FUNCTION "FC_GRP_82_R12" : VOID
TITLE =GROUP =82_R12
VERSION : 0.1


VAR_TEMP
  CL : "UDT_CABINET";	//CABINET LOCAL
  CR : "UDT_CABINET";	//CABINET REMOTE
  RelError : BOOL ;	//ERROR RELEASE
  RelErrorCL : BOOL ;	//ERROR RELEASE FROM CABINET LOCAL
  RelErrorCR : BOOL ;	//ERROR RELEASE FROM CABINET REMOTE
  RelControl : BOOL ;	//CONTROL RELEASE
  RelControlCL : BOOL ;	//CONTROL RELEASE FROM CABINET LOCAL
  RelControlCR : BOOL ;	//CONTROL RELEASE FROM CABINET REMOTE
  ErrorConfirm : BOOL ;	//ERROR CONFIRM
  AutoOn : BOOL ;	//AUTOMATIC ON
  AutoOff : BOOL ;	//AUTOMATIC OFF
  RelAuto : BOOL ;	//AUTOMATIC RELEASE
  TempSetpoint : REAL ;
  LAMP_ON : BOOL ;
  Speed_Pump_Hz : REAL ;
END_VAR
BEGIN
NETWORK
TITLE =GLOBAL SIGNALS
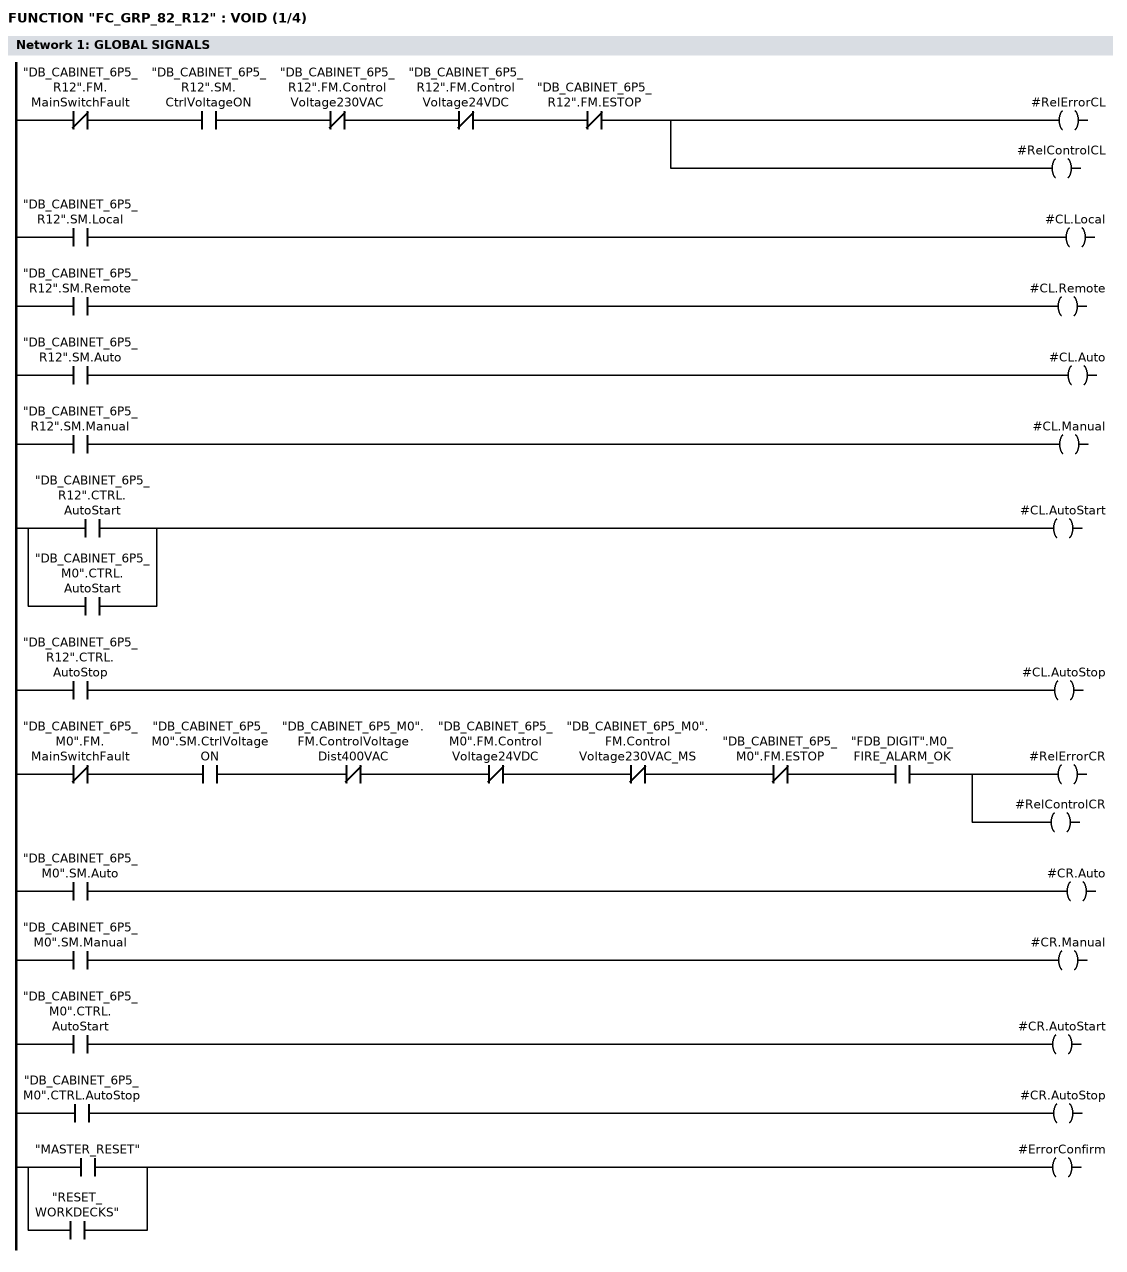
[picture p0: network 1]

      UN    "DB_CABINET_6P5_R12".FM.MainSwitchFault;
      U     "DB_CABINET_6P5_R12".SM.CtrlVoltageON;
      UN    "DB_CABINET_6P5_R12".FM.ControlVoltage230VAC;
      UN    "DB_CABINET_6P5_R12".FM.ControlVoltage24VDC;
      UN    "DB_CABINET_6P5_R12".FM.ESTOP;
      =     #RelErrorCL;
      =     #RelControlCL;

      U     "DB_CABINET_6P5_R12".SM.Local;
      =     #CL.Local;
      U     "DB_CABINET_6P5_R12".SM.Remote;
      =     #CL.Remote;
      U     "DB_CABINET_6P5_R12".SM.Auto;
      =     #CL.Auto;
      U     "DB_CABINET_6P5_R12".SM.Manual;
      =     #CL.Manual;
      U     "DB_CABINET_6P5_R12".CTRL.AutoStart;
      O     "DB_CABINET_6P5_M0".CTRL.AutoStart;
      =     #CL.AutoStart;
      U     "DB_CABINET_6P5_R12".CTRL.AutoStop;
      =     #CL.AutoStop;


      UN    "DB_CABINET_6P5_M0".FM.MainSwitchFault;
      U     "DB_CABINET_6P5_M0".SM.CtrlVoltageON;
      UN    "DB_CABINET_6P5_M0".FM.ControlVoltageDist400VAC;
      UN    "DB_CABINET_6P5_M0".FM.ControlVoltage24VDC;
      UN    "DB_CABINET_6P5_M0".FM.ControlVoltage230VAC_MS;
      UN    "DB_CABINET_6P5_M0".FM.ESTOP;
      U     "FDB_DIGIT".M0_FIRE_ALARM_OK;
      =     #RelErrorCR;
      =     #RelControlCR;

      U     "DB_CABINET_6P5_M0".SM.Auto;
      =     #CR.Auto;
      U     "DB_CABINET_6P5_M0".SM.Manual;
      =     #CR.Manual;
      U     "DB_CABINET_6P5_M0".CTRL.AutoStart;
      =     #CR.AutoStart;
      U     "DB_CABINET_6P5_M0".CTRL.AutoStop;
      =     #CR.AutoStop;


      U     "MASTER_RESET";
      O     "RESET_WORKDECKS";
      =     #ErrorConfirm;

NETWORK
TITLE =GENERAL ERROR AND WARNING
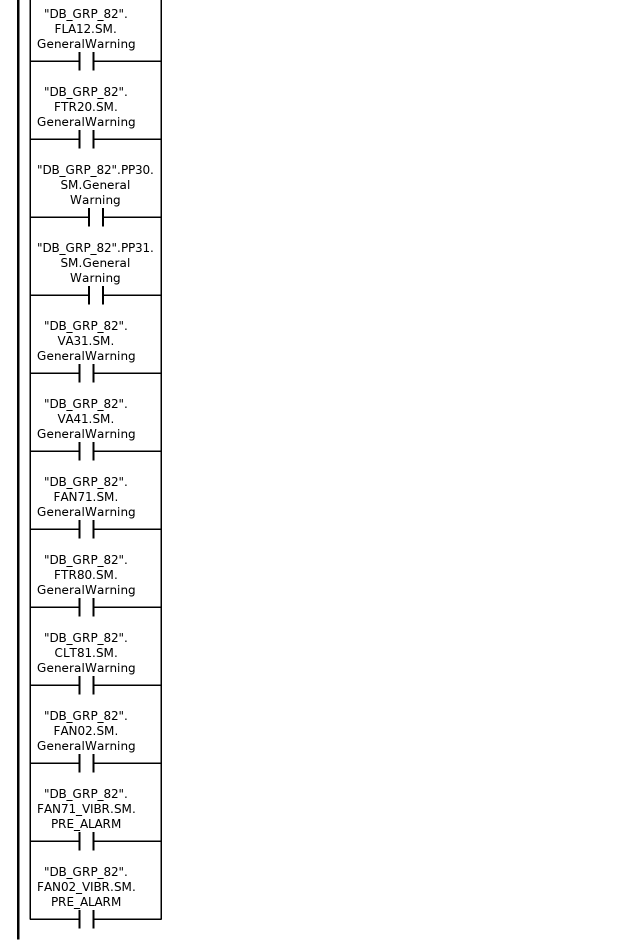
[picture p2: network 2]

      U     "DB_GRP_82".FLA11.SM.GeneralError;
      O     "DB_GRP_82".FLA12.SM.GeneralError;
      O     "DB_GRP_82".FTR20.SM.GeneralError;
      O     "DB_GRP_82".PP30.SM.GeneralError;
      O     "DB_GRP_82".PP31.SM.GeneralError;
      O     "DB_GRP_82".VA31.SM.GeneralError;
      O     "DB_GRP_82".VA41.SM.GeneralError;
      O     "DB_GRP_82".FAN71.SM.GeneralError;
      O     "DB_GRP_82".FTR80.SM.GeneralError;
      O     "DB_GRP_82".CLT81.SM.GeneralError;
      O     "DB_GRP_82".FAN02.SM.GeneralError;
      O     "DB_DIGIT".FM.GRP82_14H2_82FAN02_S32F;
      O     "DB_DIGIT".FM.GRP82_12H2_82FAN71_S32F;
      O     "DB_GRP_82".FAN71_VIBR.SM.GENERAL_ERROR;
      O     "DB_GRP_82".FAN02_VIBR.SM.GENERAL_ERROR;
      O     "DB_DIGIT".FM.GRP82_12H1_82DOO05_S90FA;
      U     "DB_PROG".WorkDecks.SM.WorkDecks2_ASU_ON;
      =     "GENERAL_FAULT_GROUP_82";


      U     "DB_GRP_82".FLA11.SM.GeneralWarning;
      O     "DB_GRP_82".FLA12.SM.GeneralWarning;
      O     "DB_GRP_82".FTR20.SM.GeneralWarning;
      O     "DB_GRP_82".PP30.SM.GeneralWarning;
      O     "DB_GRP_82".PP31.SM.GeneralWarning;
      O     "DB_GRP_82".VA31.SM.GeneralWarning;
      O     "DB_GRP_82".VA41.SM.GeneralWarning;
      O     "DB_GRP_82".FAN71.SM.GeneralWarning;
      O     "DB_GRP_82".FTR80.SM.GeneralWarning;
      O     "DB_GRP_82".CLT81.SM.GeneralWarning;
      O     "DB_GRP_82".FAN02.SM.GeneralWarning;
      O     "DB_GRP_82".FAN71_VIBR.SM.PRE_ALARM;
      O     "DB_GRP_82".FAN02_VIBR.SM.PRE_ALARM;
      =     "WARNING_GROUP_82";


NETWORK
TITLE =GENERAL ERROR 6P5_R12 (FOR LAMP AND HORN)
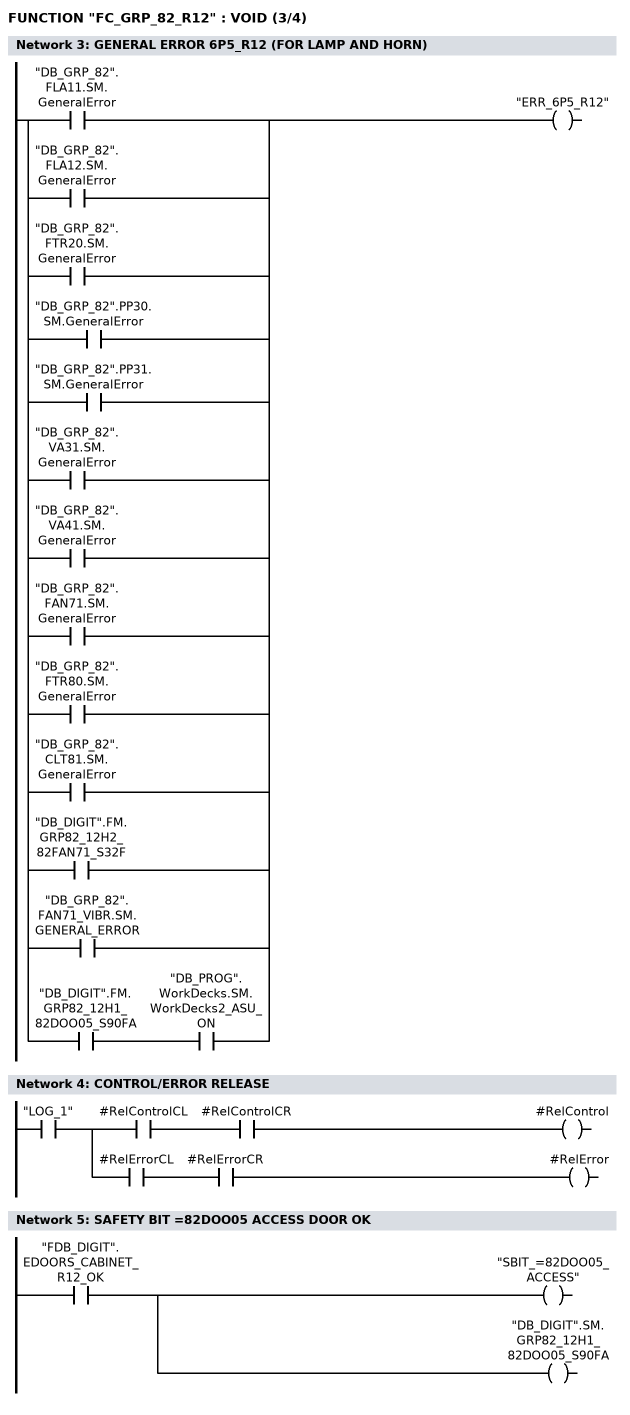
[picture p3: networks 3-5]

      O     "DB_GRP_82".FLA11.SM.GeneralError;
      O     "DB_GRP_82".FLA12.SM.GeneralError;
      O     "DB_GRP_82".FTR20.SM.GeneralError;
      O     "DB_GRP_82".PP30.SM.GeneralError;
      O     "DB_GRP_82".PP31.SM.GeneralError;
      O     "DB_GRP_82".VA31.SM.GeneralError;
      O     "DB_GRP_82".VA41.SM.GeneralError;
      O     "DB_GRP_82".FAN71.SM.GeneralError;
      O     "DB_GRP_82".FTR80.SM.GeneralError;
      O     "DB_GRP_82".CLT81.SM.GeneralError;
      O     "DB_DIGIT".FM.GRP82_12H2_82FAN71_S32F;




      O     "DB_GRP_82".FAN71_VIBR.SM.GENERAL_ERROR;
      O     ;
      U     "DB_DIGIT".FM.GRP82_12H1_82DOO05_S90FA;
      U     "DB_PROG".WorkDecks.SM.WorkDecks2_ASU_ON;
      =     "ERR_6P5_R12";
NETWORK
TITLE =CONTROL/ERROR RELEASE

      U     "LOG_1";
      =     L     16.0;
      U     L     16.0;
      U     #RelControlCL;
      U     #RelControlCR;
      =     #RelControl;
      U     L     16.0;
      U     #RelErrorCL;
      U     #RelErrorCR;
      =     #RelError;
NETWORK
TITLE =SAFETY BIT =82DOO05 ACCESS DOOR OK

      U     "FDB_DIGIT".EDOORS_CABINET_R12_OK;
      =     "SBIT_=82DOO05_ACCESS";
      =     "DB_DIGIT".SM.GRP82_12H1_82DOO05_S90FA;
NETWORK
TITLE ==82DOO05_S90FA ACCESS DOOR OK/FAULT
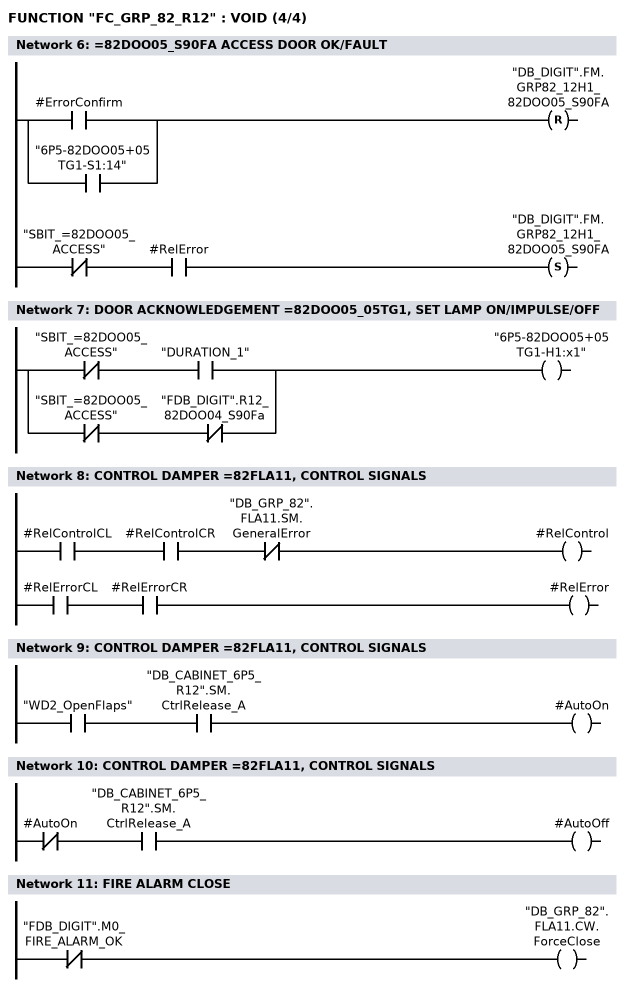
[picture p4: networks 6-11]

      U(    ;
      O     #ErrorConfirm;
      O     "6P5-82DOO05+05TG1-S1:14";
      )     ;
      R     "DB_DIGIT".FM.GRP82_12H1_82DOO05_S90FA;
      UN    "SBIT_=82DOO05_ACCESS";
      U     #RelError;
      S     "DB_DIGIT".FM.GRP82_12H1_82DOO05_S90FA;
      NOP   0;
NETWORK
TITLE =DOOR ACKNOWLEDGEMENT =82DOO05_05TG1, SET LAMP ON/IMPULSE/OFF

      UN    "SBIT_=82DOO05_ACCESS";
      U     "DURATION_1";
      O     ;
      UN    "SBIT_=82DOO05_ACCESS";
      UN    "FDB_DIGIT".R12_82DOO04_S90Fa;
      =     "6P5-82DOO05+05TG1-H1:x1";
NETWORK
TITLE =CONTROL DAMPER =82FLA11, CONTROL SIGNALS

      U     #RelControlCL;
      U     #RelControlCR;
      UN    "DB_GRP_82".FLA11.SM.GeneralError;
      =     #RelControl;

      U     #RelErrorCL;
      U     #RelErrorCR;
      =     #RelError;
NETWORK
TITLE =CONTROL DAMPER =82FLA11, CONTROL SIGNALS

      U     "WD2_OpenFlaps";
      U     "DB_CABINET_6P5_R12".SM.CtrlRelease_A;
      =     #AutoOn;
NETWORK
TITLE =CONTROL DAMPER =82FLA11, CONTROL SIGNALS

      UN    #AutoOn;
      U     "DB_CABINET_6P5_R12".SM.CtrlRelease_A;
      =     #AutoOff;
NETWORK
TITLE =FIRE ALARM CLOSE

      UN    "FDB_DIGIT".M0_FIRE_ALARM_OK;
      =     "DB_GRP_82".FLA11.CW.ForceClose;
NETWORK
TITLE =CONTROL DAMPER =82FLA11

      U     #RelControl;
      =     L     16.0;
      BLD   103;
      U     #RelError;
      =     L     16.1;
      BLD   103;
      U     #AutoOn;
      =     L     16.2;
      BLD   103;
      U     #AutoOff;
      =     L     16.3;
      BLD   103;
      U     "LOG_1";
      =     L     16.4;
      BLD   103;
      U(    ;
      U     "6P5-82FLA11+X-S1c:4";
      L     S5T#1M;
      SE    "T_Delay_Open82FLA11";
      NOP   0;
      NOP   0;
      NOP   0;
      U     "T_Delay_Open82FLA11";
      )     ;
      =     L     16.5;
      BLD   103;
      U(    ;
      U     "6P5-82FLA11+X-S2c:4";
      L     S5T#1M;
      SE    "T_Delay_Close82FLA11";
      NOP   0;
      NOP   0;
      NOP   0;
      U     "T_Delay_Close82FLA11";
      )     ;
      =     L     16.6;
      BLD   103;
      U     #ErrorConfirm;
      =     L     16.7;
      BLD   103;
      CALL "FC_FLAP" (
           REL_CONTROL              := L     16.0,
           REL_ERROR                := L     16.1,
           CL                       := #CL,
           CR                       := #CR,
           AUTO_OPEN                := L     16.2,
           AUTO_CLOSE               := L     16.3,
           FUSE                     := L     16.4,
           LS_OPEN                  := L     16.5,
           LS_CLOSE                 := L     16.6,
           ERROR_CONFIRM            := L     16.7,
           MAX_RUNTIME              := 300,
           OPEN                     := "6P5-82FLA11+X-M1:2",
           CLOSE                    := "6P5-82FLA11+X-M1:3",
           DDB                      := "DB_GRP_82".FLA11);
      NOP   0;
NETWORK
TITLE =CONTROL DAMPER =82FLA12, CONTROL SIGNALS
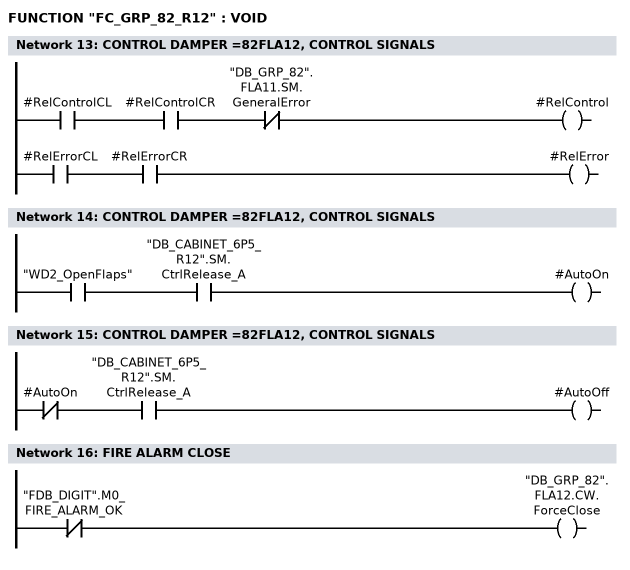
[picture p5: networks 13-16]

      U     #RelControlCL;
      U     #RelControlCR;
      UN    "DB_GRP_82".FLA11.SM.GeneralError;
      =     #RelControl;

      U     #RelErrorCL;
      U     #RelErrorCR;
      =     #RelError;



NETWORK
TITLE =CONTROL DAMPER =82FLA12, CONTROL SIGNALS

      U     "WD2_OpenFlaps";
      U     "DB_CABINET_6P5_R12".SM.CtrlRelease_A;
      =     #AutoOn;
NETWORK
TITLE =CONTROL DAMPER =82FLA12, CONTROL SIGNALS

      UN    #AutoOn;
      U     "DB_CABINET_6P5_R12".SM.CtrlRelease_A;
      =     #AutoOff;
NETWORK
TITLE =FIRE ALARM CLOSE

      UN    "FDB_DIGIT".M0_FIRE_ALARM_OK;
      =     "DB_GRP_82".FLA12.CW.ForceClose;
NETWORK
TITLE =CONTROL DAMPER =82FLA12

      U     #RelControl;
      =     L     16.0;
      BLD   103;
      U     #RelError;
      =     L     16.1;
      BLD   103;
      U     #AutoOn;
      =     L     16.2;
      BLD   103;
      U     #AutoOff;
      =     L     16.3;
      BLD   103;
      U     "LOG_1";
      =     L     16.4;
      BLD   103;
      U(    ;
      U     "6P5-82FLA12+X-S1c:4";
      L     S5T#1M;
      SE    "T_Delay_Open82FLA12";
      NOP   0;
      NOP   0;
      NOP   0;
      U     "T_Delay_Open82FLA12";
      )     ;
      =     L     16.5;
      BLD   103;
      U(    ;
      U     "6P5-82FLA12+X-S2c:4";
      L     S5T#1M;
      SE    "T_Delay_Close82FLA12";
      NOP   0;
      NOP   0;
      NOP   0;
      U     "T_Delay_Close82FLA12";
      )     ;
      =     L     16.6;
      BLD   103;
      U     #ErrorConfirm;
      =     L     16.7;
      BLD   103;
      CALL "FC_FLAP" (
           REL_CONTROL              := L     16.0,
           REL_ERROR                := L     16.1,
           CL                       := #CL,
           CR                       := #CR,
           AUTO_OPEN                := L     16.2,
           AUTO_CLOSE               := L     16.3,
           FUSE                     := L     16.4,
           LS_OPEN                  := L     16.5,
           LS_CLOSE                 := L     16.6,
           ERROR_CONFIRM            := L     16.7,
           MAX_RUNTIME              := 300,
           OPEN                     := "6P5-82FLA12+X-M1:2",
           CLOSE                    := "6P5-82FLA12+X-M1:3",
           DDB                      := "DB_GRP_82".FLA12);
      NOP   0;
NETWORK
TITLE =FILTER MONITOR =82FTR20-B33
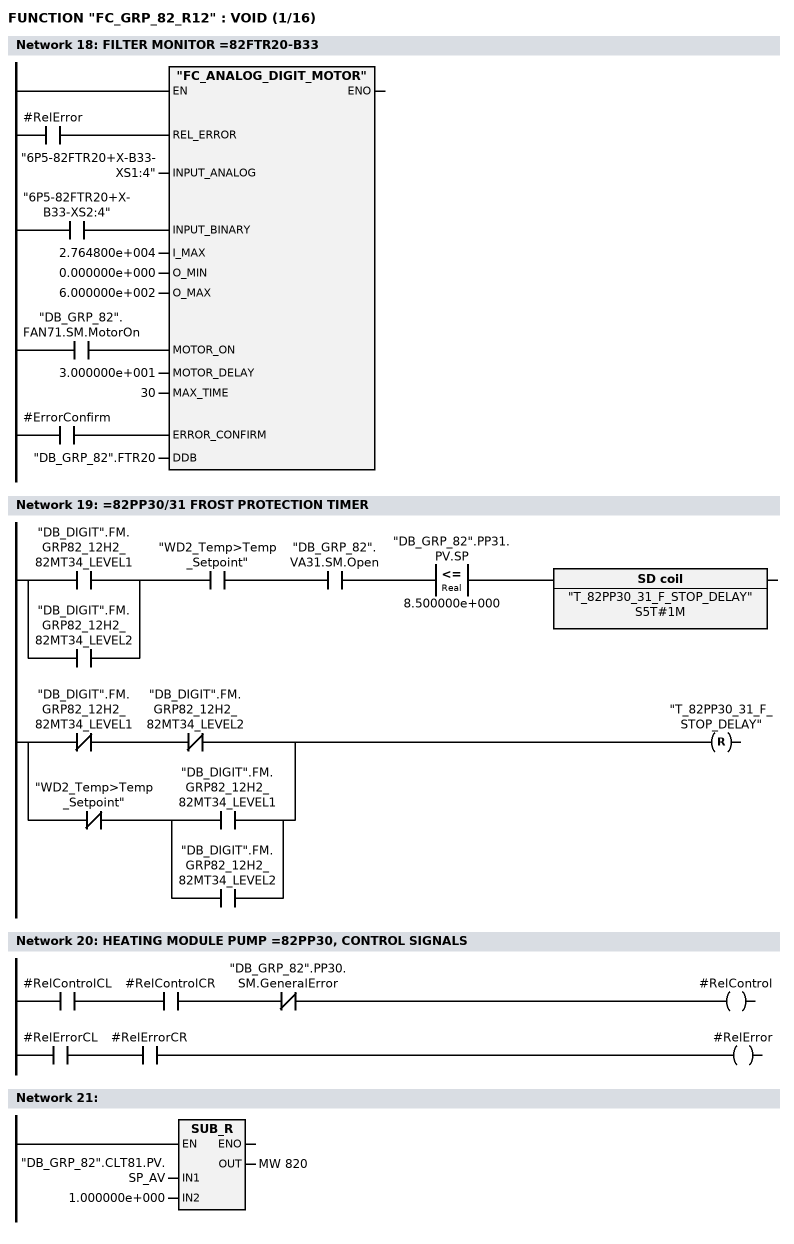
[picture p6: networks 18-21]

      U     #RelError;
      =     L     16.0;
      BLD   103;
      U     "6P5-82FTR20+X-B33-XS2:4";
      =     L     16.1;
      BLD   103;
      U     "DB_GRP_82".FAN71.SM.MotorOn;
      =     L     16.2;
      BLD   103;
      U     #ErrorConfirm;
      =     L     16.3;
      BLD   103;
      CALL "FC_ANALOG_DIGIT_MOTOR" (
           REL_ERROR                := L     16.0,
           INPUT_ANALOG             := "6P5-82FTR20+X-B33-XS1:4",
           INPUT_BINARY             := L     16.1,
           I_MAX                    := 2.764800e+004,
           O_MIN                    := 0.000000e+000,
           O_MAX                    := 6.000000e+002,
           MOTOR_ON                 := L     16.2,
           MOTOR_DELAY              := 3.000000e+001,
           MAX_TIME                 := 30,
           ERROR_CONFIRM            := L     16.3,
           DDB                      := "DB_GRP_82".FTR20);
      NOP   0;
NETWORK
TITLE ==82PP30/31 FROST PROTECTION TIMER

      U(    ;
      O     "DB_DIGIT".FM.GRP82_12H2_82MT34_LEVEL1;
      O     "DB_DIGIT".FM.GRP82_12H2_82MT34_LEVEL2;
      )     ;
      U     "WD2_Temp>Temp_Setpoint";
      U     "DB_GRP_82".VA31.SM.Open;
      U(    ;
      L     "DB_GRP_82".PP31.PV.SP;
      L     8.500000e+000;
      <=R   ;
      )     ;
      L     S5T#1M;
      SE    "T_82PP30_31_F_STOP_DELAY";
      U(    ;
      UN    "DB_DIGIT".FM.GRP82_12H2_82MT34_LEVEL1;
      UN    "DB_DIGIT".FM.GRP82_12H2_82MT34_LEVEL2;
      O     ;
      UN    "WD2_Temp>Temp_Setpoint";
      U(    ;
      O     "DB_DIGIT".FM.GRP82_12H2_82MT34_LEVEL1;
      O     "DB_DIGIT".FM.GRP82_12H2_82MT34_LEVEL2;
      )     ;
      )     ;
      R     "T_82PP30_31_F_STOP_DELAY";
      NOP   0;
      NOP   0;
      NOP   0;
NETWORK
TITLE =HEATING MODULE PUMP =82PP30, CONTROL SIGNALS

      U     #RelControlCL;
      U     #RelControlCR;
      UN    "DB_GRP_82".PP30.SM.GeneralError;
      =     #RelControl;

      U     #RelErrorCL;
      U     #RelErrorCR;
      =     #RelError;

NETWORK
TITLE =

      L     "DB_GRP_82".CLT81.PV.SP_AV;
      L     1.000000e+000;
      -R    ;
      T     MW   820;
      NOP   0;
NETWORK
TITLE =AUTO ON
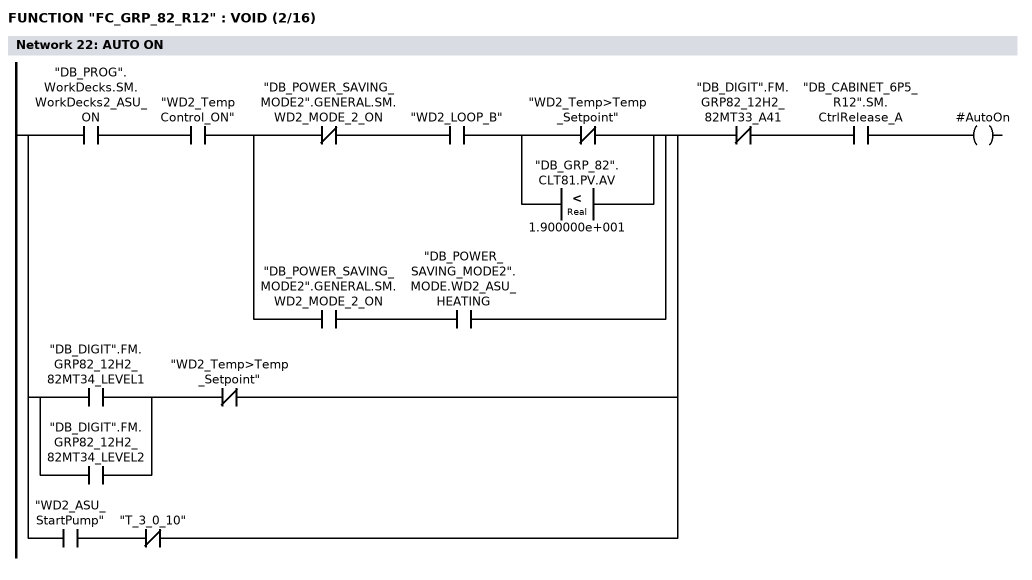
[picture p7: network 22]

      U(    ;
      U     "DB_PROG".WorkDecks.SM.WorkDecks2_ASU_ON;
      U     "WD2_TempControl_ON";
      U(    ;
      UN    "DB_POWER_SAVING_MODE2".GENERAL.SM.WD2_MODE_2_ON;
      U     "WD2_LOOP_B";
      U(    ;
      ON    "WD2_Temp>Temp_Setpoint";
      O(    ;
      L     "DB_GRP_82".CLT81.PV.AV;
      L     1.900000e+001;
      <R    ;
      )     ;
      )     ;
      O     ;
      U     "DB_POWER_SAVING_MODE2".GENERAL.SM.WD2_MODE_2_ON;
      U     "DB_POWER_SAVING_MODE2".MODE.WD2_ASU_HEATING;
      )     ;
      O     ;
      U(    ;
      O     "DB_DIGIT".FM.GRP82_12H2_82MT34_LEVEL1;
      O     "DB_DIGIT".FM.GRP82_12H2_82MT34_LEVEL2;
      )     ;
      UN    "WD2_Temp>Temp_Setpoint";
      O     ;
      U     "WD2_ASU_StartPump";
      UN    "T_3_0_10";
      )     ;
      UN    "DB_DIGIT".FM.GRP82_12H2_82MT33_A41;
      U     "DB_CABINET_6P5_R12".SM.CtrlRelease_A;
      =     #AutoOn;
NETWORK
TITLE =AUTO OFF
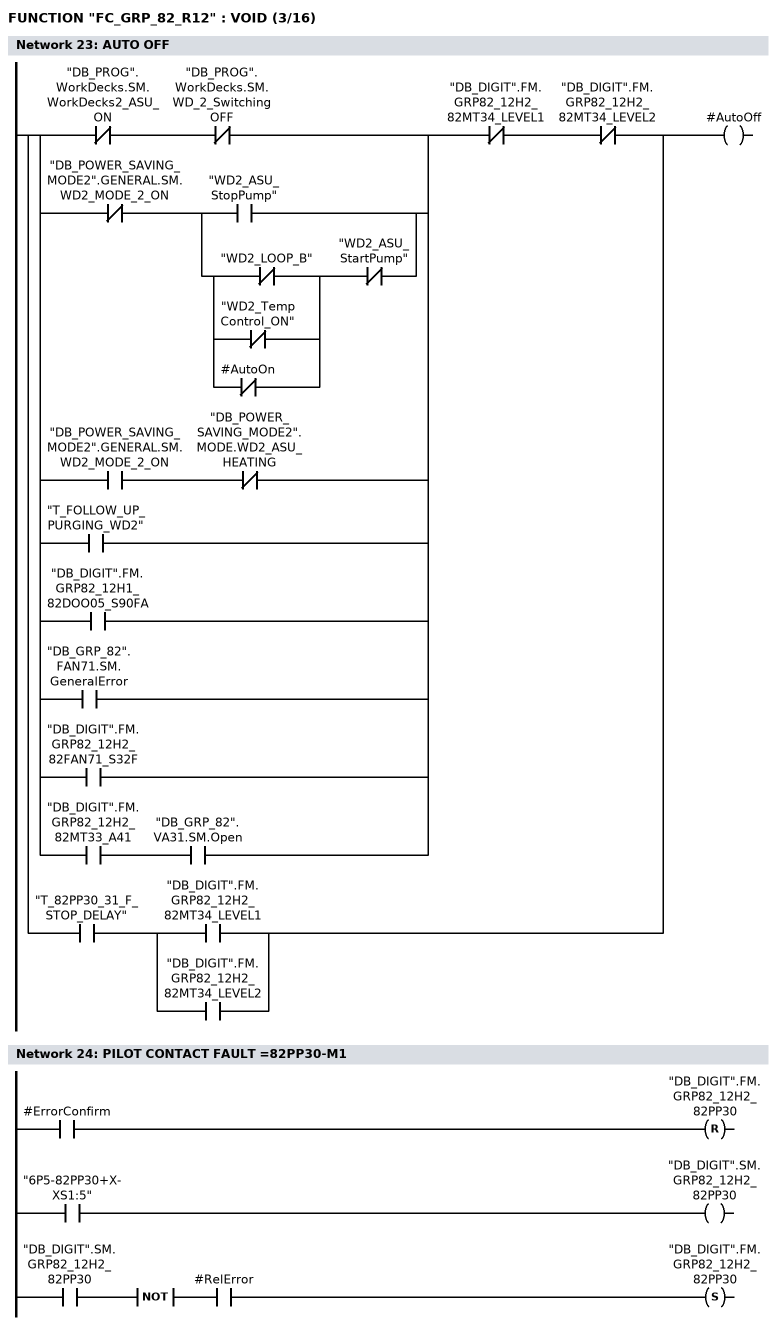
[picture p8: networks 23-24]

      U(    ;
      UN    "DB_PROG".WorkDecks.SM.WorkDecks2_ASU_ON;
      UN    "DB_PROG".WorkDecks.SM.WD_2_SwitchingOFF;
      O     ;
      UN    "DB_POWER_SAVING_MODE2".GENERAL.SM.WD2_MODE_2_ON;
      U(    ;
      O     "WD2_ASU_StopPump";
      O     ;
      U(    ;
      ON    "WD2_LOOP_B";
      ON    "WD2_TempControl_ON";
      ON    #AutoOn;
      )     ;
      UN    "WD2_ASU_StartPump";
      )     ;
      O     ;
      U     "DB_POWER_SAVING_MODE2".GENERAL.SM.WD2_MODE_2_ON;
      UN    "DB_POWER_SAVING_MODE2".MODE.WD2_ASU_HEATING;
      O     "T_FOLLOW_UP_PURGING_WD2";
      O     "DB_DIGIT".FM.GRP82_12H1_82DOO05_S90FA;
      O     "DB_GRP_82".FAN71.SM.GeneralError;
      O     "DB_DIGIT".FM.GRP82_12H2_82FAN71_S32F;
      O     ;
      U     "DB_DIGIT".FM.GRP82_12H2_82MT33_A41;
      U     "DB_GRP_82".VA31.SM.Open;
      )     ;
      UN    "DB_DIGIT".FM.GRP82_12H2_82MT34_LEVEL1;
      UN    "DB_DIGIT".FM.GRP82_12H2_82MT34_LEVEL2;
      O     ;
      U     "T_82PP30_31_F_STOP_DELAY";
      U(    ;
      O     "DB_DIGIT".FM.GRP82_12H2_82MT34_LEVEL1;
      O     "DB_DIGIT".FM.GRP82_12H2_82MT34_LEVEL2;
      )     ;
      =     #AutoOff;
NETWORK
TITLE =PILOT CONTACT FAULT =82PP30-M1

      U     #ErrorConfirm;
      R     "DB_DIGIT".FM.GRP82_12H2_82PP30;
      U     "6P5-82PP30+X-XS1:5";
      =     "DB_DIGIT".SM.GRP82_12H2_82PP30;
      U     "DB_DIGIT".SM.GRP82_12H2_82PP30;
      NOT   ;
      U     #RelError;
      S     "DB_DIGIT".FM.GRP82_12H2_82PP30;
      NOP   0;
NETWORK
TITLE =HEATING MODULE PUMP, =82PP30-M1
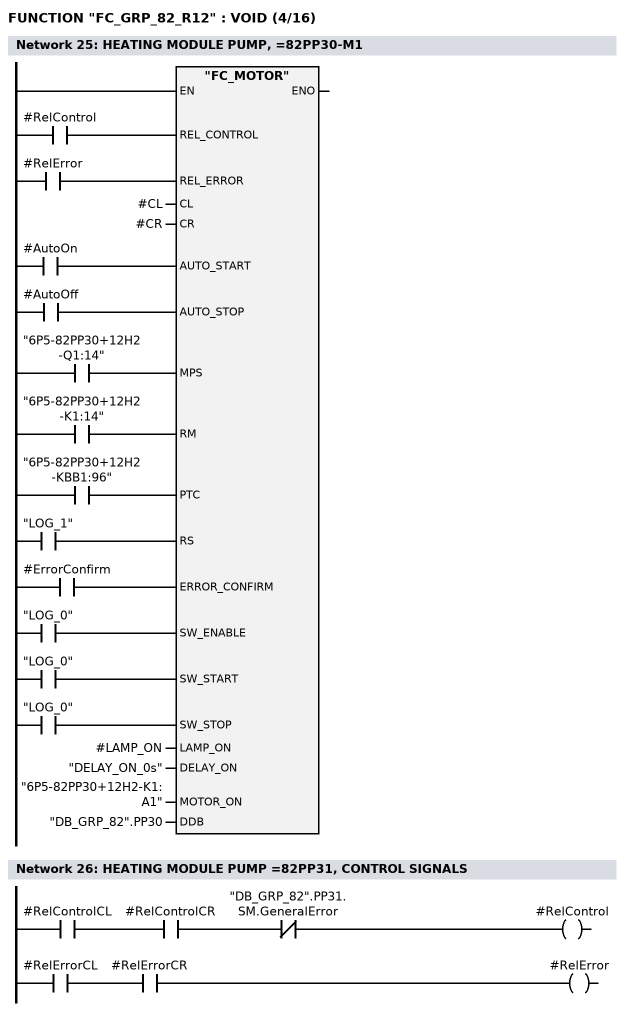
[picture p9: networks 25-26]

      U     #RelControl;
      =     L     16.0;
      BLD   103;
      U     #RelError;
      =     L     16.1;
      BLD   103;
      U     #AutoOn;
      =     L     16.2;
      BLD   103;
      U     #AutoOff;
      =     L     16.3;
      BLD   103;
      U     "6P5-82PP30+12H2-Q1:14";
      =     L     16.4;
      BLD   103;
      U     "6P5-82PP30+12H2-K1:14";
      =     L     16.5;
      BLD   103;
      U     "6P5-82PP30+12H2-KBB1:96";
      =     L     16.6;
      BLD   103;
      U     "LOG_1";
      =     L     16.7;
      BLD   103;
      U     #ErrorConfirm;
      =     L     17.0;
      BLD   103;
      U     "LOG_0";
      =     L     17.1;
      BLD   103;
      U     "LOG_0";
      =     L     17.2;
      BLD   103;
      U     "LOG_0";
      =     L     17.3;
      BLD   103;
      CALL "FC_MOTOR" (
           REL_CONTROL              := L     16.0,
           REL_ERROR                := L     16.1,
           CL                       := #CL,
           CR                       := #CR,
           AUTO_START               := L     16.2,
           AUTO_STOP                := L     16.3,
           MPS                      := L     16.4,
           RM                       := L     16.5,
           PTC                      := L     16.6,
           RS                       := L     16.7,
           ERROR_CONFIRM            := L     17.0,
           SW_ENABLE                := L     17.1,
           SW_START                 := L     17.2,
           SW_STOP                  := L     17.3,
           LAMP_ON                  := #LAMP_ON,
           DELAY_ON                 := "DELAY_ON_0s",
           MOTOR_ON                 := "6P5-82PP30+12H2-K1:A1",
           DDB                      := "DB_GRP_82".PP30);
      NOP   0;
NETWORK
TITLE =HEATING MODULE PUMP =82PP31, CONTROL SIGNALS

      U     #RelControlCL;
      U     #RelControlCR;
      UN    "DB_GRP_82".PP31.SM.GeneralError;
      =     #RelControl;

      U     #RelErrorCL;
      U     #RelErrorCR;
      =     #RelError;



NETWORK
TITLE =AUTO ON
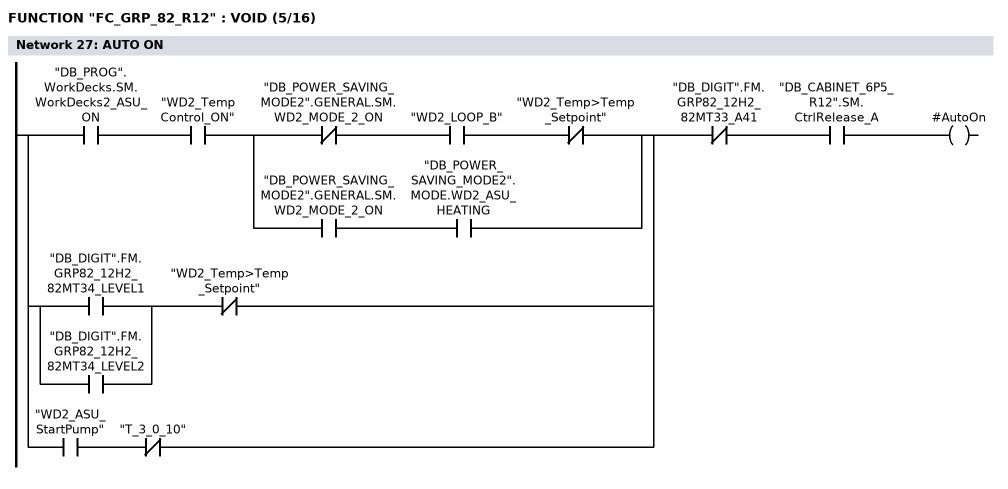
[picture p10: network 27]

      U(    ;
      U     "DB_PROG".WorkDecks.SM.WorkDecks2_ASU_ON;
      U     "WD2_TempControl_ON";
      U(    ;
      UN    "DB_POWER_SAVING_MODE2".GENERAL.SM.WD2_MODE_2_ON;
      U     "WD2_LOOP_B";
      UN    "WD2_Temp>Temp_Setpoint";
      O     ;
      U     "DB_POWER_SAVING_MODE2".GENERAL.SM.WD2_MODE_2_ON;
      U     "DB_POWER_SAVING_MODE2".MODE.WD2_ASU_HEATING;
      )     ;
      O     ;
      U(    ;
      O     "DB_DIGIT".FM.GRP82_12H2_82MT34_LEVEL1;
      O     "DB_DIGIT".FM.GRP82_12H2_82MT34_LEVEL2;
      )     ;
      UN    "WD2_Temp>Temp_Setpoint";
      O     ;
      U     "WD2_ASU_StartPump";
      UN    "T_3_0_10";
      )     ;
      UN    "DB_DIGIT".FM.GRP82_12H2_82MT33_A41;
      U     "DB_CABINET_6P5_R12".SM.CtrlRelease_A;
      =     #AutoOn;
NETWORK
TITLE =AUTO OFF
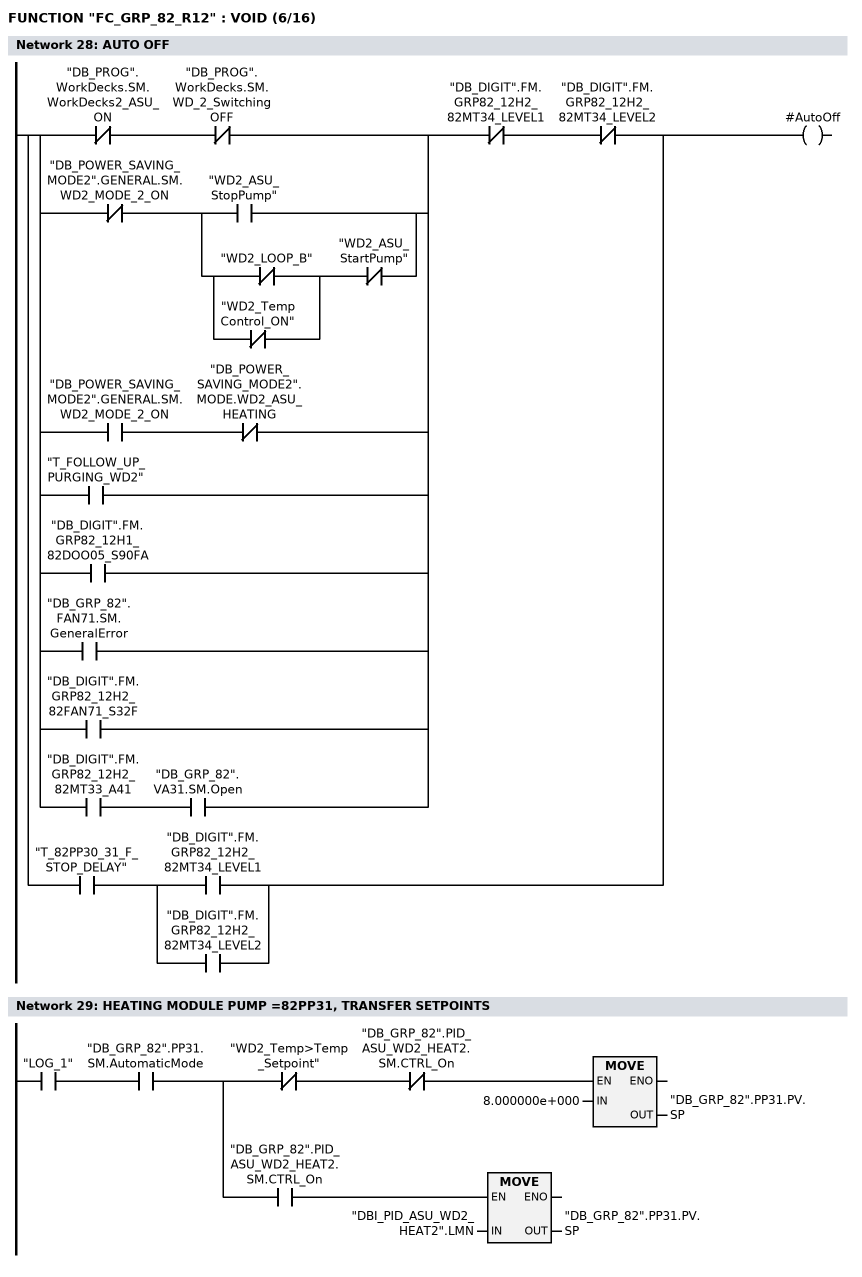
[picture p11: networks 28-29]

      U(    ;
      UN    "DB_PROG".WorkDecks.SM.WorkDecks2_ASU_ON;
      UN    "DB_PROG".WorkDecks.SM.WD_2_SwitchingOFF;
      O     ;
      UN    "DB_POWER_SAVING_MODE2".GENERAL.SM.WD2_MODE_2_ON;
      U(    ;
      O     "WD2_ASU_StopPump";
      O     ;
      U(    ;
      ON    "WD2_LOOP_B";
      ON    "WD2_TempControl_ON";
      )     ;
      UN    "WD2_ASU_StartPump";
      )     ;
      O     ;
      U     "DB_POWER_SAVING_MODE2".GENERAL.SM.WD2_MODE_2_ON;
      UN    "DB_POWER_SAVING_MODE2".MODE.WD2_ASU_HEATING;
      O     "T_FOLLOW_UP_PURGING_WD2";
      O     "DB_DIGIT".FM.GRP82_12H1_82DOO05_S90FA;
      O     "DB_GRP_82".FAN71.SM.GeneralError;
      O     "DB_DIGIT".FM.GRP82_12H2_82FAN71_S32F;
      O     ;
      U     "DB_DIGIT".FM.GRP82_12H2_82MT33_A41;
      U     "DB_GRP_82".VA31.SM.Open;
      )     ;
      UN    "DB_DIGIT".FM.GRP82_12H2_82MT34_LEVEL1;
      UN    "DB_DIGIT".FM.GRP82_12H2_82MT34_LEVEL2;
      O     ;
      U     "T_82PP30_31_F_STOP_DELAY";
      U(    ;
      O     "DB_DIGIT".FM.GRP82_12H2_82MT34_LEVEL1;
      O     "DB_DIGIT".FM.GRP82_12H2_82MT34_LEVEL2;
      )     ;
      =     #AutoOff;
NETWORK
TITLE =HEATING MODULE PUMP =82PP31, TRANSFER SETPOINTS

      U     "LOG_1";
      U     "DB_GRP_82".PP31.SM.AutomaticMode;
      =     L     16.0;
      U     L     16.0;
      UN    "WD2_Temp>Temp_Setpoint";
      UN    "DB_GRP_82".PID_ASU_WD2_HEAT2.SM.CTRL_On;
      SPBNB _001;
      L     8.000000e+000;
      T     "DB_GRP_82".PP31.PV.SP;
_001: NOP   0;
      U     L     16.0;
      U     "DB_GRP_82".PID_ASU_WD2_HEAT2.SM.CTRL_On;
      SPBNB _002;
      L     "DBI_PID_ASU_WD2_HEAT2".LMN;
      T     "DB_GRP_82".PP31.PV.SP;
_002: NOP   0;
NETWORK
TITLE =HEATING MODULE PUMP, =82PP31_M1
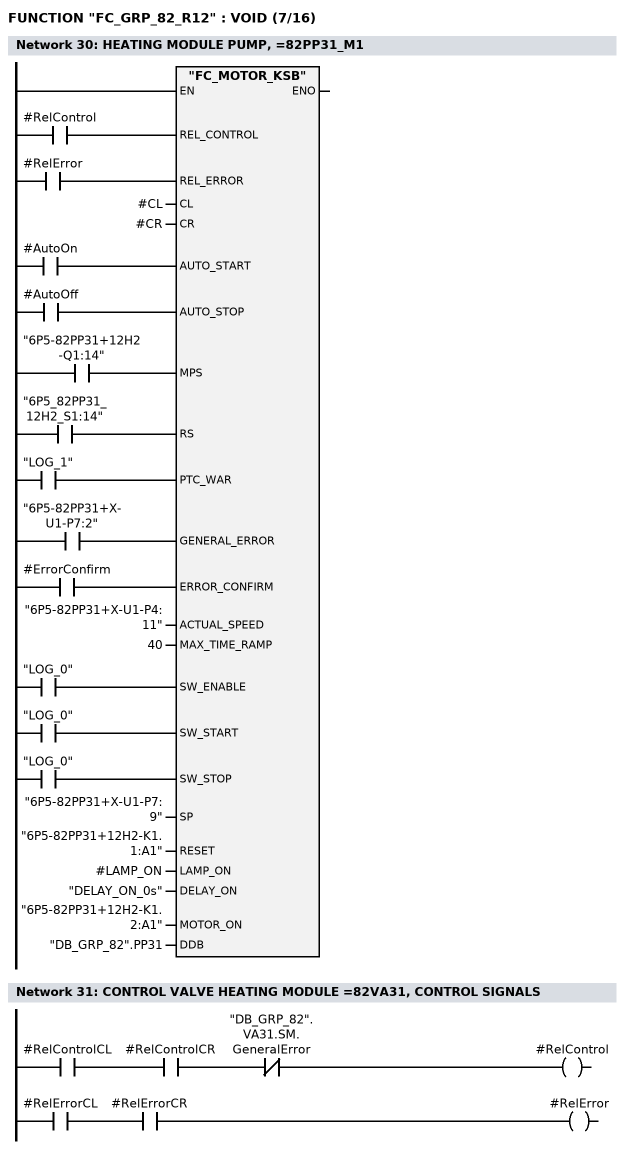
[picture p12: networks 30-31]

      U     #RelControl;
      =     L     16.0;
      BLD   103;
      U     #RelError;
      =     L     16.1;
      BLD   103;
      U     #AutoOn;
      =     L     16.2;
      BLD   103;
      U     #AutoOff;
      =     L     16.3;
      BLD   103;
      U     "6P5-82PP31+12H2-Q1:14";
      =     L     16.4;
      BLD   103;
      U     "6P5_82PP31_12H2_S1:14";
      =     L     16.5;
      BLD   103;
      U     "LOG_1";
      =     L     16.6;
      BLD   103;
      U     "6P5-82PP31+X-U1-P7:2";
      =     L     16.7;
      BLD   103;
      U     #ErrorConfirm;
      =     L     17.0;
      BLD   103;
      U     "LOG_0";
      =     L     17.1;
      BLD   103;
      U     "LOG_0";
      =     L     17.2;
      BLD   103;
      U     "LOG_0";
      =     L     17.3;
      BLD   103;
      CALL "FC_MOTOR_KSB" (
           REL_CONTROL              := L     16.0,
           REL_ERROR                := L     16.1,
           CL                       := #CL,
           CR                       := #CR,
           AUTO_START               := L     16.2,
           AUTO_STOP                := L     16.3,
           MPS                      := L     16.4,
           RS                       := L     16.5,
           PTC_WAR                  := L     16.6,
           GENERAL_ERROR            := L     16.7,
           ERROR_CONFIRM            := L     17.0,
           ACTUAL_SPEED             := "6P5-82PP31+X-U1-P4:11",
           MAX_TIME_RAMP            := 40,
           SW_ENABLE                := L     17.1,
           SW_START                 := L     17.2,
           SW_STOP                  := L     17.3,
           SP                       := "6P5-82PP31+X-U1-P7:9",
           RESET                    := "6P5-82PP31+12H2-K1.1:A1",
           LAMP_ON                  := #LAMP_ON,
           DELAY_ON                 := "DELAY_ON_0s",
           MOTOR_ON                 := "6P5-82PP31+12H2-K1.2:A1",
           DDB                      := "DB_GRP_82".PP31);
      NOP   0;
NETWORK
TITLE =CONTROL VALVE HEATING MODULE =82VA31, CONTROL SIGNALS

      U     #RelControlCL;
      U     #RelControlCR;
      UN    "DB_GRP_82".VA31.SM.GeneralError;
      =     #RelControl;

      U     #RelErrorCL;
      U     #RelErrorCR;
      =     #RelError;
NETWORK
TITLE =AUTO ON
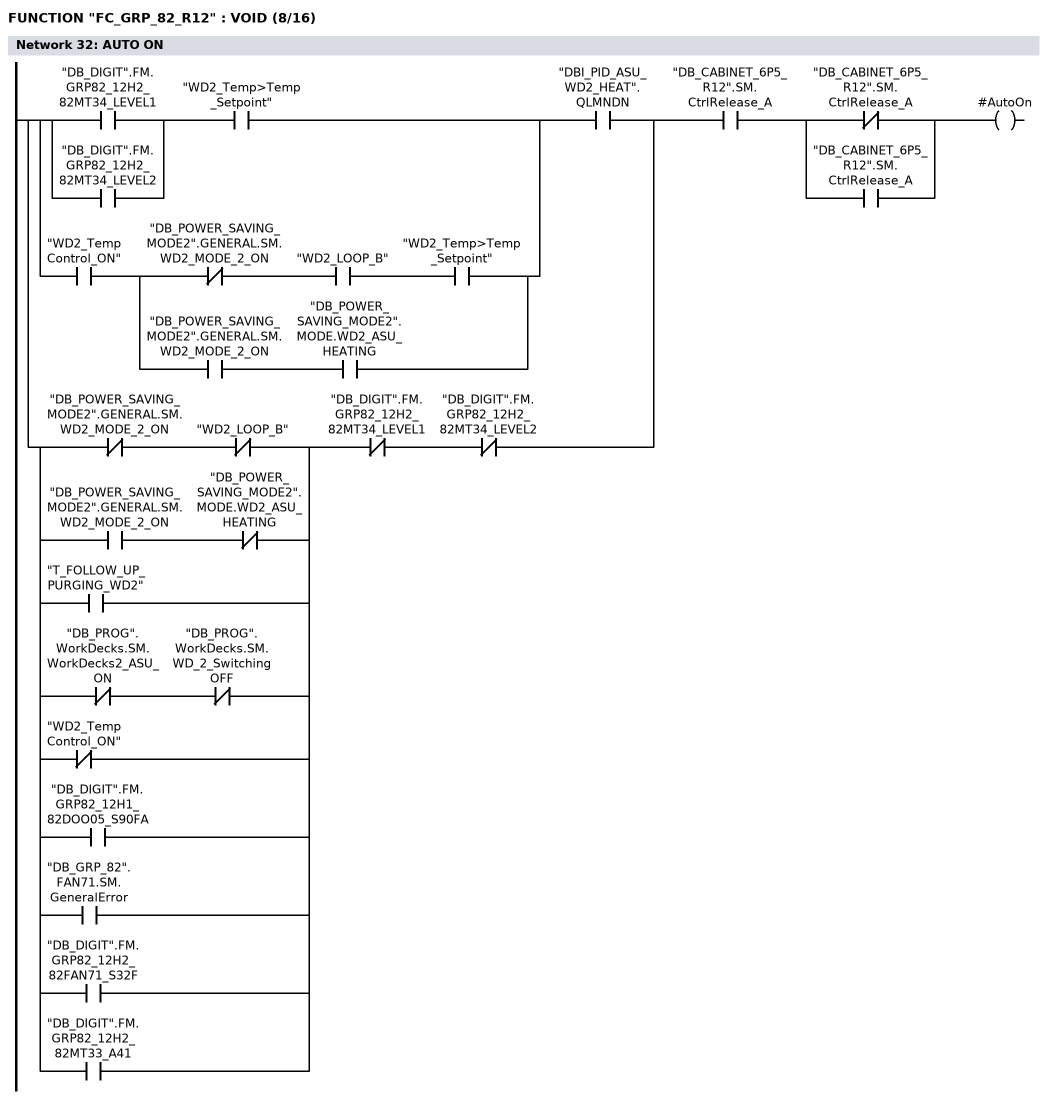
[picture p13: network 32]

      U(    ;
      U(    ;
      U(    ;
      O     "DB_DIGIT".FM.GRP82_12H2_82MT34_LEVEL1;
      O     "DB_DIGIT".FM.GRP82_12H2_82MT34_LEVEL2;
      )     ;
      U     "WD2_Temp>Temp_Setpoint";
      O     ;
      U     "WD2_TempControl_ON";
      U(    ;
      UN    "DB_POWER_SAVING_MODE2".GENERAL.SM.WD2_MODE_2_ON;
      U     "WD2_LOOP_B";
      U     "WD2_Temp>Temp_Setpoint";
      O     ;
      U     "DB_POWER_SAVING_MODE2".GENERAL.SM.WD2_MODE_2_ON;
      U     "DB_POWER_SAVING_MODE2".MODE.WD2_ASU_HEATING;
      )     ;
      )     ;
      U     "DBI_PID_ASU_WD2_HEAT".QLMNDN;
      O     ;
      U(    ;
      UN    "DB_POWER_SAVING_MODE2".GENERAL.SM.WD2_MODE_2_ON;
      UN    "WD2_LOOP_B";
      O     ;
      U     "DB_POWER_SAVING_MODE2".GENERAL.SM.WD2_MODE_2_ON;
      UN    "DB_POWER_SAVING_MODE2".MODE.WD2_ASU_HEATING;
      O     "T_FOLLOW_UP_PURGING_WD2";
      O     ;
      UN    "DB_PROG".WorkDecks.SM.WorkDecks2_ASU_ON;
      UN    "DB_PROG".WorkDecks.SM.WD_2_SwitchingOFF;
      ON    "WD2_TempControl_ON";
      O     "DB_DIGIT".FM.GRP82_12H1_82DOO05_S90FA;
      O     "DB_GRP_82".FAN71.SM.GeneralError;
      O     "DB_DIGIT".FM.GRP82_12H2_82FAN71_S32F;
      O     "DB_DIGIT".FM.GRP82_12H2_82MT33_A41;
      )     ;
      UN    "DB_DIGIT".FM.GRP82_12H2_82MT34_LEVEL1;
      UN    "DB_DIGIT".FM.GRP82_12H2_82MT34_LEVEL2;
      )     ;
      U     "DB_CABINET_6P5_R12".SM.CtrlRelease_A;
      U(    ;
      ON    "DB_CABINET_6P5_R12".SM.CtrlRelease_A;
      O     "DB_CABINET_6P5_R12".SM.CtrlRelease_A;
      )     ;
      =     #AutoOn;
NETWORK
TITLE =AUTO OFF
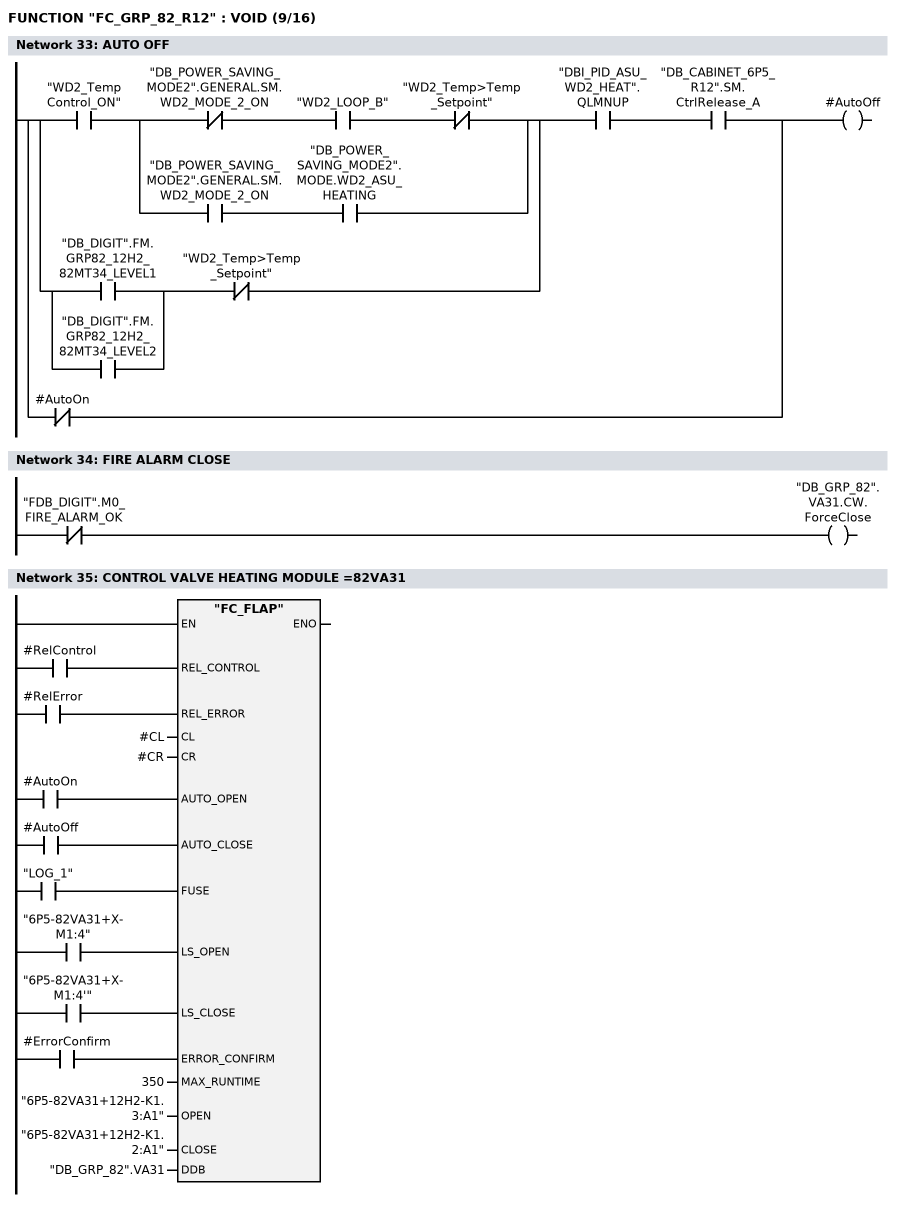
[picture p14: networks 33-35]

      U(    ;
      U     "WD2_TempControl_ON";
      U(    ;
      UN    "DB_POWER_SAVING_MODE2".GENERAL.SM.WD2_MODE_2_ON;
      U     "WD2_LOOP_B";
      UN    "WD2_Temp>Temp_Setpoint";
      O     ;
      U     "DB_POWER_SAVING_MODE2".GENERAL.SM.WD2_MODE_2_ON;
      U     "DB_POWER_SAVING_MODE2".MODE.WD2_ASU_HEATING;
      )     ;
      O     ;
      U(    ;
      O     "DB_DIGIT".FM.GRP82_12H2_82MT34_LEVEL1;
      O     "DB_DIGIT".FM.GRP82_12H2_82MT34_LEVEL2;
      )     ;
      UN    "WD2_Temp>Temp_Setpoint";
      )     ;
      U     "DBI_PID_ASU_WD2_HEAT".QLMNUP;
      U     "DB_CABINET_6P5_R12".SM.CtrlRelease_A;
      ON    #AutoOn;
      =     #AutoOff;
NETWORK
TITLE =FIRE ALARM CLOSE

      UN    "FDB_DIGIT".M0_FIRE_ALARM_OK;
      =     "DB_GRP_82".VA31.CW.ForceClose;
NETWORK
TITLE =CONTROL VALVE HEATING MODULE =82VA31

      U     #RelControl;
      =     L     16.0;
      BLD   103;
      U     #RelError;
      =     L     16.1;
      BLD   103;
      U     #AutoOn;
      =     L     16.2;
      BLD   103;
      U     #AutoOff;
      =     L     16.3;
      BLD   103;
      U     "LOG_1";
      =     L     16.4;
      BLD   103;
      U     "6P5-82VA31+X-M1:4";
      =     L     16.5;
      BLD   103;
      U     "6P5-82VA31+X-M1:4'";
      =     L     16.6;
      BLD   103;
      U     #ErrorConfirm;
      =     L     16.7;
      BLD   103;
      CALL "FC_FLAP" (
           REL_CONTROL              := L     16.0,
           REL_ERROR                := L     16.1,
           CL                       := #CL,
           CR                       := #CR,
           AUTO_OPEN                := L     16.2,
           AUTO_CLOSE               := L     16.3,
           FUSE                     := L     16.4,
           LS_OPEN                  := L     16.5,
           LS_CLOSE                 := L     16.6,
           ERROR_CONFIRM            := L     16.7,
           MAX_RUNTIME              := 350,
           OPEN                     := "6P5-82VA31+12H2-K1.3:A1",
           CLOSE                    := "6P5-82VA31+12H2-K1.2:A1",
           DDB                      := "DB_GRP_82".VA31);
      NOP   0;
NETWORK
TITLE =READ POSITION =82VA31
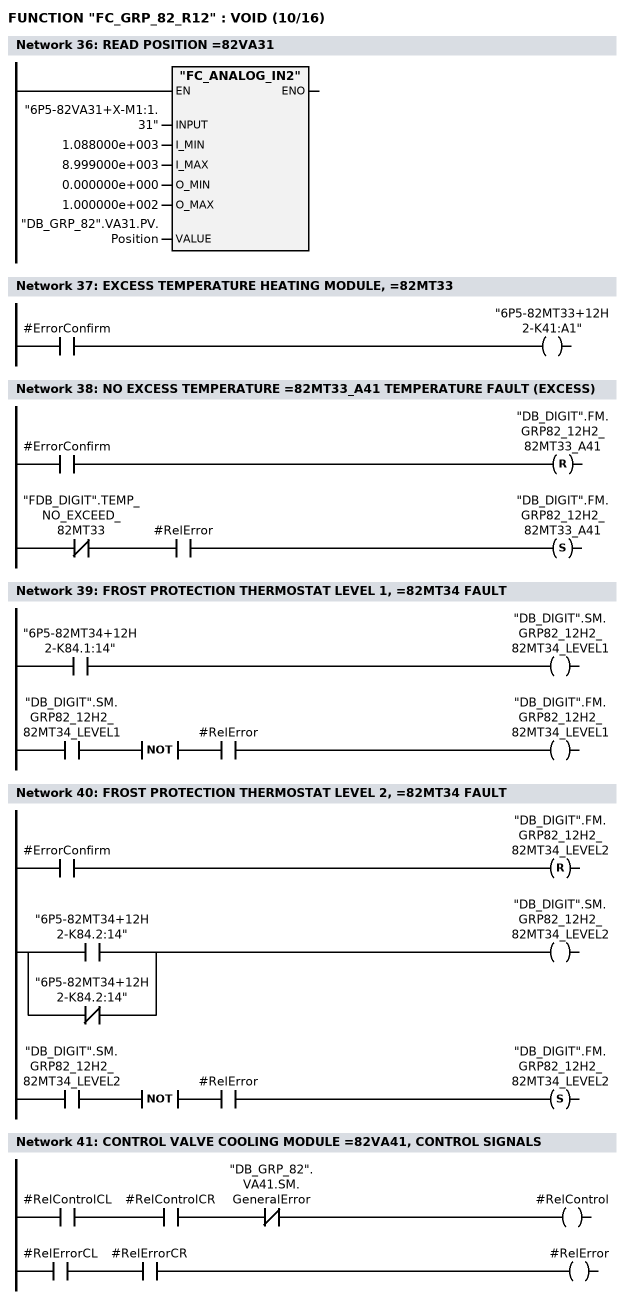
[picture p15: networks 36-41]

      CALL "FC_ANALOG_IN2" (
           INPUT                    := "6P5-82VA31+X-M1:1.31",
           I_MIN                    := 1.088000e+003,
           I_MAX                    := 8.999000e+003,
           O_MIN                    := 0.000000e+000,
           O_MAX                    := 1.000000e+002,
           VALUE                    := "DB_GRP_82".VA31.PV.Position);
      NOP   0;
NETWORK
TITLE =EXCESS TEMPERATURE HEATING MODULE, =82MT33

      U     #ErrorConfirm;
      =     "6P5-82MT33+12H2-K41:A1";
NETWORK
TITLE =NO EXCESS TEMPERATURE =82MT33_A41 TEMPERATURE FAULT (EXCESS)

      U     #ErrorConfirm;
      R     "DB_DIGIT".FM.GRP82_12H2_82MT33_A41;
      UN    "FDB_DIGIT".TEMP_NO_EXCEED_82MT33;
      U     #RelError;
      S     "DB_DIGIT".FM.GRP82_12H2_82MT33_A41;
      NOP   0;
NETWORK
TITLE =FROST PROTECTION THERMOSTAT LEVEL 1, =82MT34 FAULT

      U     "6P5-82MT34+12H2-K84.1:14";
      =     "DB_DIGIT".SM.GRP82_12H2_82MT34_LEVEL1;
      U     "DB_DIGIT".SM.GRP82_12H2_82MT34_LEVEL1;
      NOT   ;
      U     #RelError;
      =     "DB_DIGIT".FM.GRP82_12H2_82MT34_LEVEL1;
NETWORK
TITLE =FROST PROTECTION THERMOSTAT LEVEL 2, =82MT34 FAULT

      U     #ErrorConfirm;
      R     "DB_DIGIT".FM.GRP82_12H2_82MT34_LEVEL2;
      U(    ;
      O     "6P5-82MT34+12H2-K84.2:14";
      ON    "6P5-82MT34+12H2-K84.2:14";
      )     ;
      =     "DB_DIGIT".SM.GRP82_12H2_82MT34_LEVEL2;
      U     "DB_DIGIT".SM.GRP82_12H2_82MT34_LEVEL2;
      NOT   ;
      U     #RelError;
      S     "DB_DIGIT".FM.GRP82_12H2_82MT34_LEVEL2;
      NOP   0;
NETWORK
TITLE =CONTROL VALVE COOLING MODULE =82VA41, CONTROL SIGNALS

      U     #RelControlCL;
      U     #RelControlCR;
      UN    "DB_GRP_82".VA41.SM.GeneralError;
      =     #RelControl;

      U     #RelErrorCL;
      U     #RelErrorCR;
      =     #RelError;


NETWORK
TITLE =RELEASE =82VA41
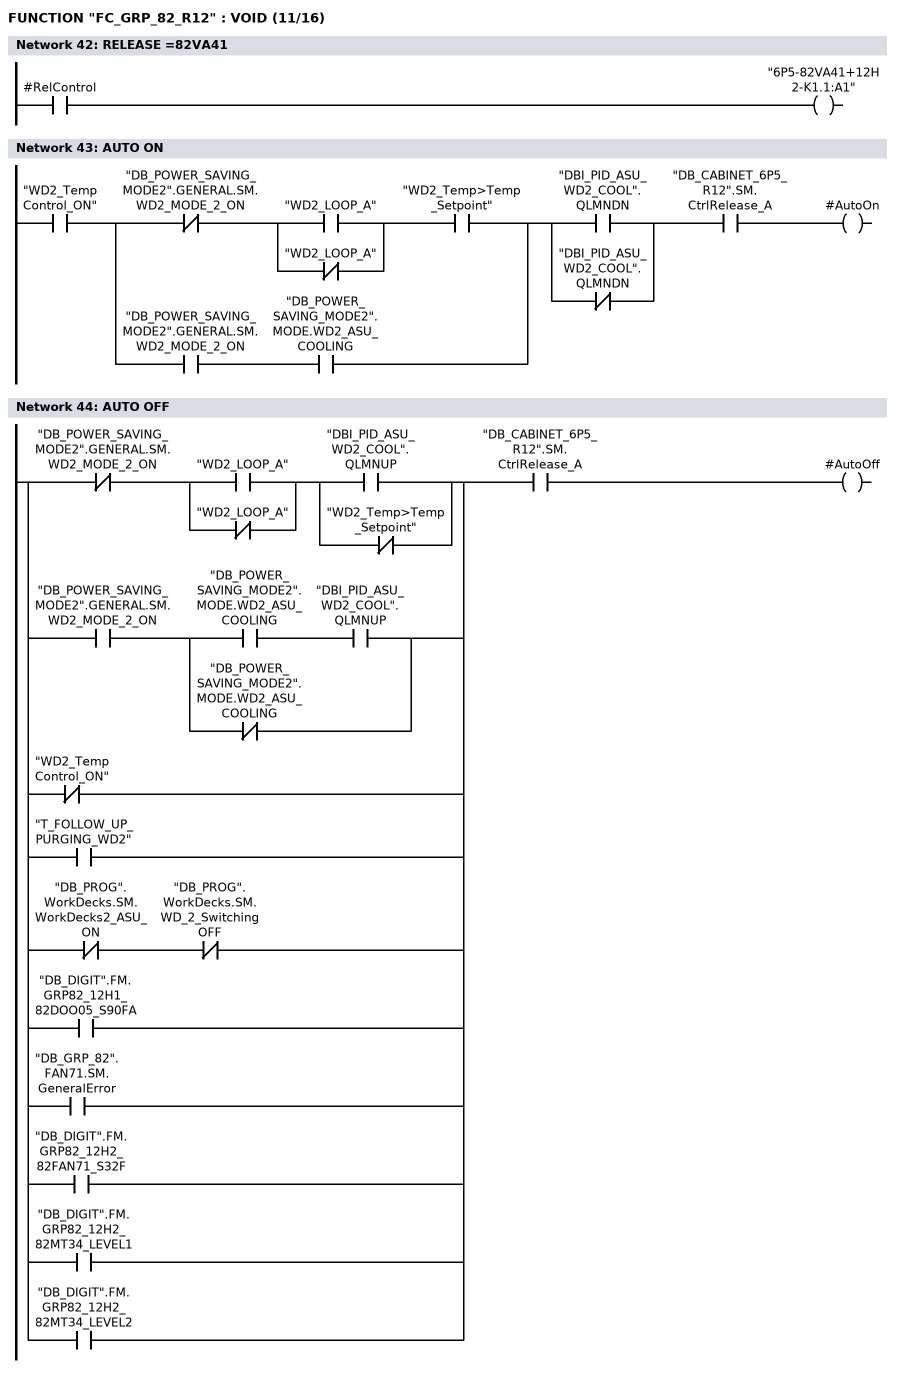
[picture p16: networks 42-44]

      U     #RelControl;
      =     "6P5-82VA41+12H2-K1.1:A1";
NETWORK
TITLE =AUTO ON

      U     "WD2_TempControl_ON";
      U(    ;
      UN    "DB_POWER_SAVING_MODE2".GENERAL.SM.WD2_MODE_2_ON;
      U(    ;
      O     "WD2_LOOP_A";
      ON    "WD2_LOOP_A";
      )     ;
      U     "WD2_Temp>Temp_Setpoint";
      O     ;
      U     "DB_POWER_SAVING_MODE2".GENERAL.SM.WD2_MODE_2_ON;
      U     "DB_POWER_SAVING_MODE2".MODE.WD2_ASU_COOLING;
      )     ;
      U(    ;
      O     "DBI_PID_ASU_WD2_COOL".QLMNDN;
      ON    "DBI_PID_ASU_WD2_COOL".QLMNDN;
      )     ;
      U     "DB_CABINET_6P5_R12".SM.CtrlRelease_A;
      =     #AutoOn;
NETWORK
TITLE =AUTO OFF

      U(    ;
      UN    "DB_POWER_SAVING_MODE2".GENERAL.SM.WD2_MODE_2_ON;
      U(    ;
      O     "WD2_LOOP_A";
      ON    "WD2_LOOP_A";
      )     ;
      U(    ;
      O     "DBI_PID_ASU_WD2_COOL".QLMNUP;
      ON    "WD2_Temp>Temp_Setpoint";
      )     ;
      O     ;
      U     "DB_POWER_SAVING_MODE2".GENERAL.SM.WD2_MODE_2_ON;
      U(    ;
      U     "DB_POWER_SAVING_MODE2".MODE.WD2_ASU_COOLING;
      U     "DBI_PID_ASU_WD2_COOL".QLMNUP;
      ON    "DB_POWER_SAVING_MODE2".MODE.WD2_ASU_COOLING;
      )     ;
      ON    "WD2_TempControl_ON";
      O     "T_FOLLOW_UP_PURGING_WD2";
      O     ;
      UN    "DB_PROG".WorkDecks.SM.WorkDecks2_ASU_ON;
      UN    "DB_PROG".WorkDecks.SM.WD_2_SwitchingOFF;
      O     "DB_DIGIT".FM.GRP82_12H1_82DOO05_S90FA;
      O     "DB_GRP_82".FAN71.SM.GeneralError;
      O     "DB_DIGIT".FM.GRP82_12H2_82FAN71_S32F;
      O     "DB_DIGIT".FM.GRP82_12H2_82MT34_LEVEL1;
      O     "DB_DIGIT".FM.GRP82_12H2_82MT34_LEVEL2;
      )     ;
      U     "DB_CABINET_6P5_R12".SM.CtrlRelease_A;
      =     #AutoOff;
NETWORK
TITLE =FIRE ALARM CLOSE
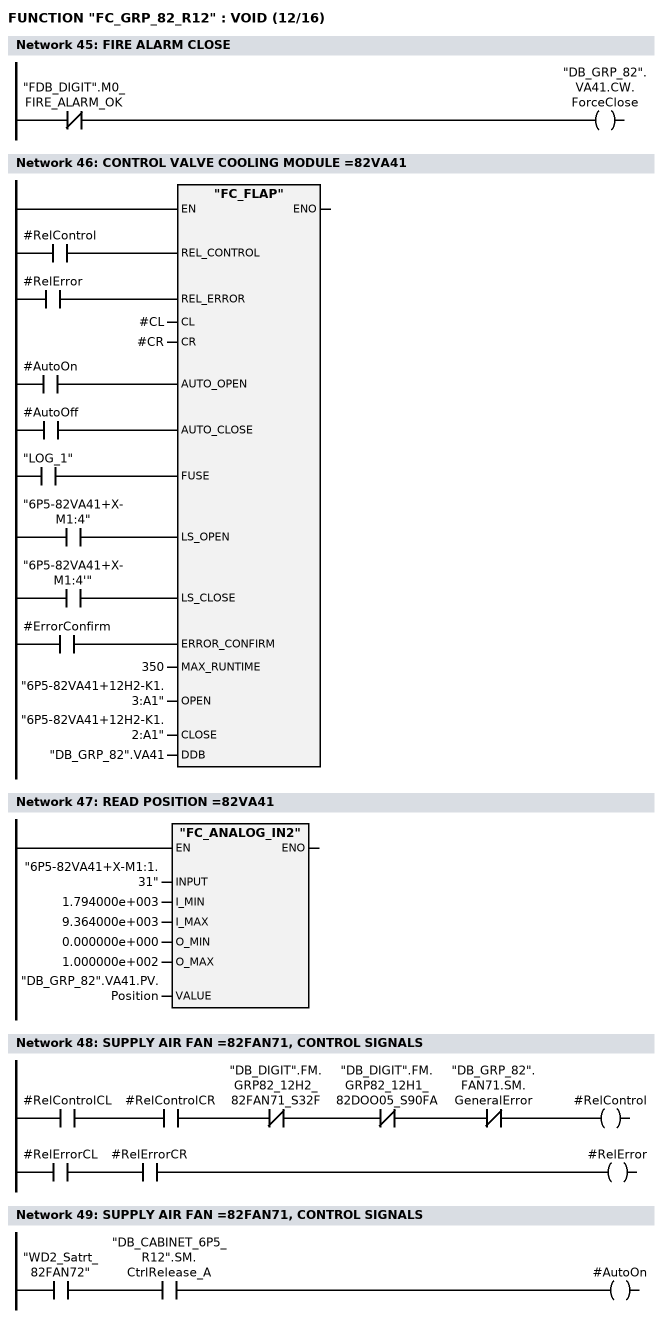
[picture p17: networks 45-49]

      UN    "FDB_DIGIT".M0_FIRE_ALARM_OK;
      =     "DB_GRP_82".VA41.CW.ForceClose;
NETWORK
TITLE =CONTROL VALVE COOLING MODULE =82VA41

      U     #RelControl;
      =     L     16.0;
      BLD   103;
      U     #RelError;
      =     L     16.1;
      BLD   103;
      U     #AutoOn;
      =     L     16.2;
      BLD   103;
      U     #AutoOff;
      =     L     16.3;
      BLD   103;
      U     "LOG_1";
      =     L     16.4;
      BLD   103;
      U     "6P5-82VA41+X-M1:4";
      =     L     16.5;
      BLD   103;
      U     "6P5-82VA41+X-M1:4'";
      =     L     16.6;
      BLD   103;
      U     #ErrorConfirm;
      =     L     16.7;
      BLD   103;
      CALL "FC_FLAP" (
           REL_CONTROL              := L     16.0,
           REL_ERROR                := L     16.1,
           CL                       := #CL,
           CR                       := #CR,
           AUTO_OPEN                := L     16.2,
           AUTO_CLOSE               := L     16.3,
           FUSE                     := L     16.4,
           LS_OPEN                  := L     16.5,
           LS_CLOSE                 := L     16.6,
           ERROR_CONFIRM            := L     16.7,
           MAX_RUNTIME              := 350,
           OPEN                     := "6P5-82VA41+12H2-K1.3:A1",
           CLOSE                    := "6P5-82VA41+12H2-K1.2:A1",
           DDB                      := "DB_GRP_82".VA41);
      NOP   0;
NETWORK
TITLE =READ POSITION =82VA41

      CALL "FC_ANALOG_IN2" (
           INPUT                    := "6P5-82VA41+X-M1:1.31",
           I_MIN                    := 1.794000e+003,
           I_MAX                    := 9.364000e+003,
           O_MIN                    := 0.000000e+000,
           O_MAX                    := 1.000000e+002,
           VALUE                    := "DB_GRP_82".VA41.PV.Position);
      NOP   0;
NETWORK
TITLE =SUPPLY AIR FAN =82FAN71, CONTROL SIGNALS

      U     #RelControlCL;
      U     #RelControlCR;
      UN    "DB_DIGIT".FM.GRP82_12H2_82FAN71_S32F;
      UN    "DB_DIGIT".FM.GRP82_12H1_82DOO05_S90FA;
      UN    "DB_GRP_82".FAN71.SM.GeneralError;
      =     #RelControl;

      U     #RelErrorCL;
      U     #RelErrorCR;
      =     #RelError;



NETWORK
TITLE =SUPPLY AIR FAN =82FAN71, CONTROL SIGNALS

      U     "WD2_Satrt_82FAN72";
      U     "DB_CABINET_6P5_R12".SM.CtrlRelease_A;
      =     #AutoOn;
NETWORK
TITLE =SUPPLY AIR FAN =82FAN71, CONTROL SIGNALS
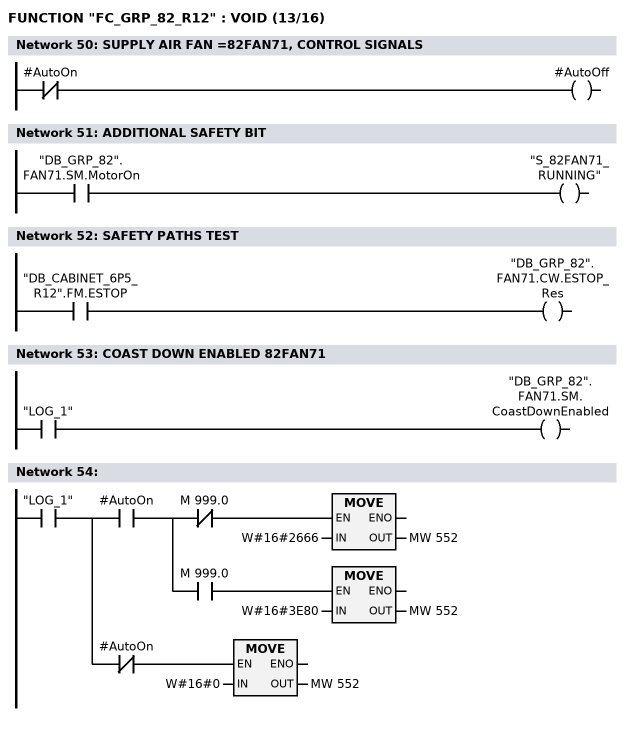
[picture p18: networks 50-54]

      UN    #AutoOn;
      =     #AutoOff;
NETWORK
TITLE =ADDITIONAL SAFETY BIT

      U     "DB_GRP_82".FAN71.SM.MotorOn;
      =     "S_82FAN71_RUNNING";
NETWORK
TITLE =SAFETY PATHS TEST

      U     "DB_CABINET_6P5_R12".FM.ESTOP;
      =     "DB_GRP_82".FAN71.CW.ESTOP_Res;
NETWORK
TITLE =COAST DOWN ENABLED 82FAN71

      U     "LOG_1";
      =     "DB_GRP_82".FAN71.SM.CoastDownEnabled;
NETWORK
TITLE =

      U     "LOG_1";
      =     L     16.0;
      U     L     16.0;
      U     #AutoOn;
      =     L     16.1;
      U     L     16.1;
      UN    M    999.0;
      SPBNB _003;
      L     W#16#2666;
      T     MW   552;
_003: NOP   0;
      U     L     16.1;
      U     M    999.0;
      SPBNB _004;
      L     W#16#3E80;
      T     MW   552;
_004: NOP   0;
      U     L     16.0;
      UN    #AutoOn;
      SPBNB _005;
      L     W#16#0;
      T     MW   552;
_005: NOP   0;
NETWORK
TITLE =SUPPLY AIR FAN =82FAN71_M1
//PEW 6072 ingresso da inserire su FC_FREQ_AV
//W#16#2666
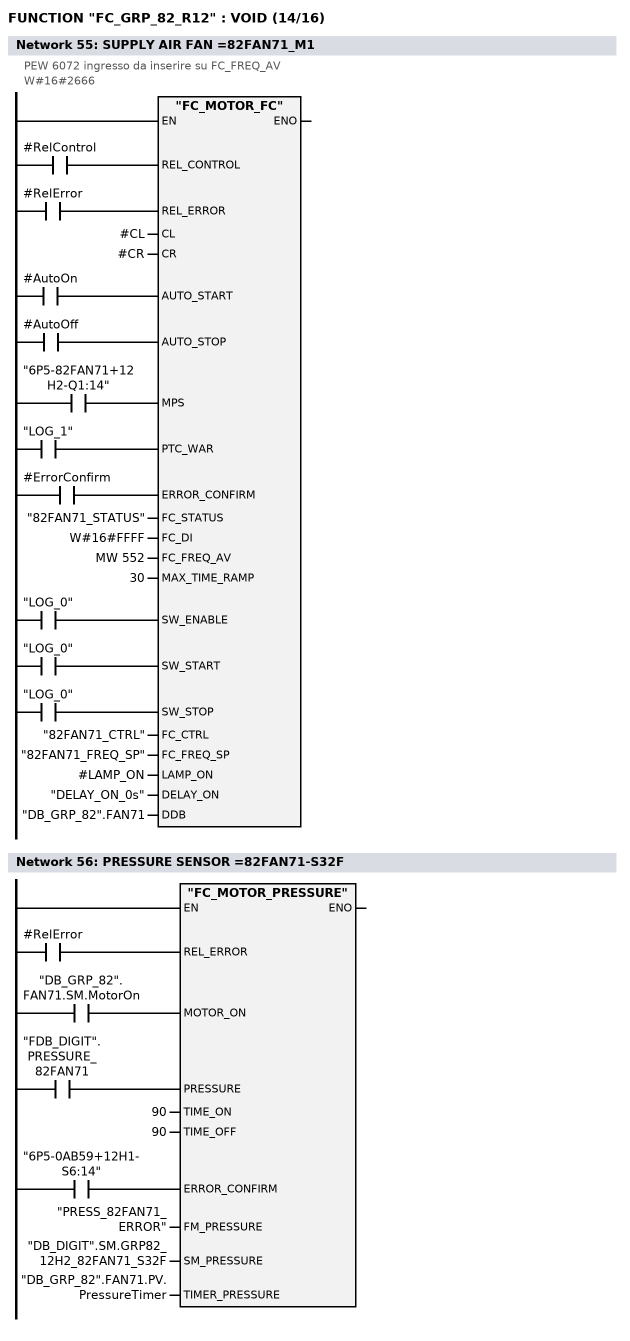
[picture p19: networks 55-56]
      U     #RelControl;
      =     L     16.0;
      BLD   103;
      U     #RelError;
      =     L     16.1;
      BLD   103;
      U     #AutoOn;
      =     L     16.2;
      BLD   103;
      U     #AutoOff;
      =     L     16.3;
      BLD   103;
      U     "6P5-82FAN71+12H2-Q1:14";
      =     L     16.4;
      BLD   103;
      U     "LOG_1";
      =     L     16.5;
      BLD   103;
      U     #ErrorConfirm;
      =     L     16.6;
      BLD   103;
      U     "LOG_0";
      =     L     16.7;
      BLD   103;
      U     "LOG_0";
      =     L     17.0;
      BLD   103;
      U     "LOG_0";
      =     L     17.1;
      BLD   103;
      CALL "FC_MOTOR_FC" (
           REL_CONTROL              := L     16.0,
           REL_ERROR                := L     16.1,
           CL                       := #CL,
           CR                       := #CR,
           AUTO_START               := L     16.2,
           AUTO_STOP                := L     16.3,
           MPS                      := L     16.4,
           PTC_WAR                  := L     16.5,
           ERROR_CONFIRM            := L     16.6,
           FC_STATUS                := "82FAN71_STATUS",
           FC_DI                    := W#16#FFFF,
           FC_FREQ_AV               := MW   552,
           MAX_TIME_RAMP            := 30,
           SW_ENABLE                := L     16.7,
           SW_START                 := L     17.0,
           SW_STOP                  := L     17.1,
           FC_CTRL                  := "82FAN71_CTRL",
           FC_FREQ_SP               := "82FAN71_FREQ_SP",
           LAMP_ON                  := #LAMP_ON,
           DELAY_ON                 := "DELAY_ON_0s",
           DDB                      := "DB_GRP_82".FAN71);
      NOP   0;
NETWORK
TITLE =PRESSURE SENSOR =82FAN71-S32F

      U     #RelError;
      =     L     16.0;
      BLD   103;
      U     "DB_GRP_82".FAN71.SM.MotorOn;
      =     L     16.1;
      BLD   103;
      U     "FDB_DIGIT".PRESSURE_82FAN71;
      =     L     16.2;
      BLD   103;
      U     "6P5-0AB59+12H1-S6:14";
      =     L     16.3;
      BLD   103;
      CALL "FC_MOTOR_PRESSURE" (
           REL_ERROR                := L     16.0,
           MOTOR_ON                 := L     16.1,
           PRESSURE                 := L     16.2,
           TIME_ON                  := 90,
           TIME_OFF                 := 90,
           ERROR_CONFIRM            := L     16.3,
           FM_PRESSURE              := "PRESS_82FAN71_ERROR",
           SM_PRESSURE              := "DB_DIGIT".SM.GRP82_12H2_82FAN71_S32F,
           TIMER_PRESSURE           := "DB_GRP_82".FAN71.PV.PressureTimer);
      NOP   0;
NETWORK
TITLE =PRESSURE ERROR =82FAN71
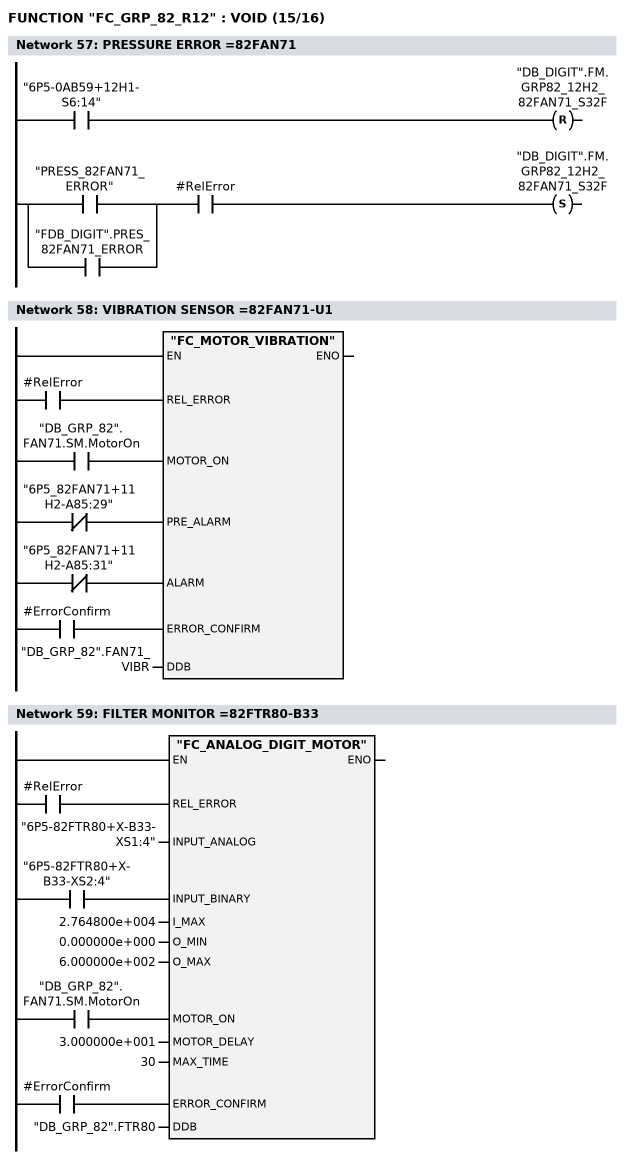
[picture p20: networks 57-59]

      U     "6P5-0AB59+12H1-S6:14";
      R     "DB_DIGIT".FM.GRP82_12H2_82FAN71_S32F;
      U(    ;
      O     "PRESS_82FAN71_ERROR";
      O     "FDB_DIGIT".PRES_82FAN71_ERROR;
      )     ;
      U     #RelError;
      S     "DB_DIGIT".FM.GRP82_12H2_82FAN71_S32F;
      NOP   0;
NETWORK
TITLE =VIBRATION SENSOR =82FAN71-U1

      U     #RelError;
      =     L     16.0;
      BLD   103;
      U     "DB_GRP_82".FAN71.SM.MotorOn;
      =     L     16.1;
      BLD   103;
      UN    "6P5_82FAN71+11H2-A85:29";
      =     L     16.2;
      BLD   103;
      UN    "6P5_82FAN71+11H2-A85:31";
      =     L     16.3;
      BLD   103;
      U     #ErrorConfirm;
      =     L     16.4;
      BLD   103;
      CALL "FC_MOTOR_VIBRATION" (
           REL_ERROR                := L     16.0,
           MOTOR_ON                 := L     16.1,
           PRE_ALARM                := L     16.2,
           ALARM                    := L     16.3,
           ERROR_CONFIRM            := L     16.4,
           DDB                      := "DB_GRP_82".FAN71_VIBR);
      NOP   0;
NETWORK
TITLE =FILTER MONITOR =82FTR80-B33

      U     #RelError;
      =     L     16.0;
      BLD   103;
      U     "6P5-82FTR80+X-B33-XS2:4";
      =     L     16.1;
      BLD   103;
      U     "DB_GRP_82".FAN71.SM.MotorOn;
      =     L     16.2;
      BLD   103;
      U     #ErrorConfirm;
      =     L     16.3;
      BLD   103;
      CALL "FC_ANALOG_DIGIT_MOTOR" (
           REL_ERROR                := L     16.0,
           INPUT_ANALOG             := "6P5-82FTR80+X-B33-XS1:4",
           INPUT_BINARY             := L     16.1,
           I_MAX                    := 2.764800e+004,
           O_MIN                    := 0.000000e+000,
           O_MAX                    := 6.000000e+002,
           MOTOR_ON                 := L     16.2,
           MOTOR_DELAY              := 3.000000e+001,
           MAX_TIME                 := 30,
           ERROR_CONFIRM            := L     16.3,
           DDB                      := "DB_GRP_82".FTR80);
      NOP   0;
NETWORK
TITLE ==82CLT81-B40N SETPOINT CHANGED
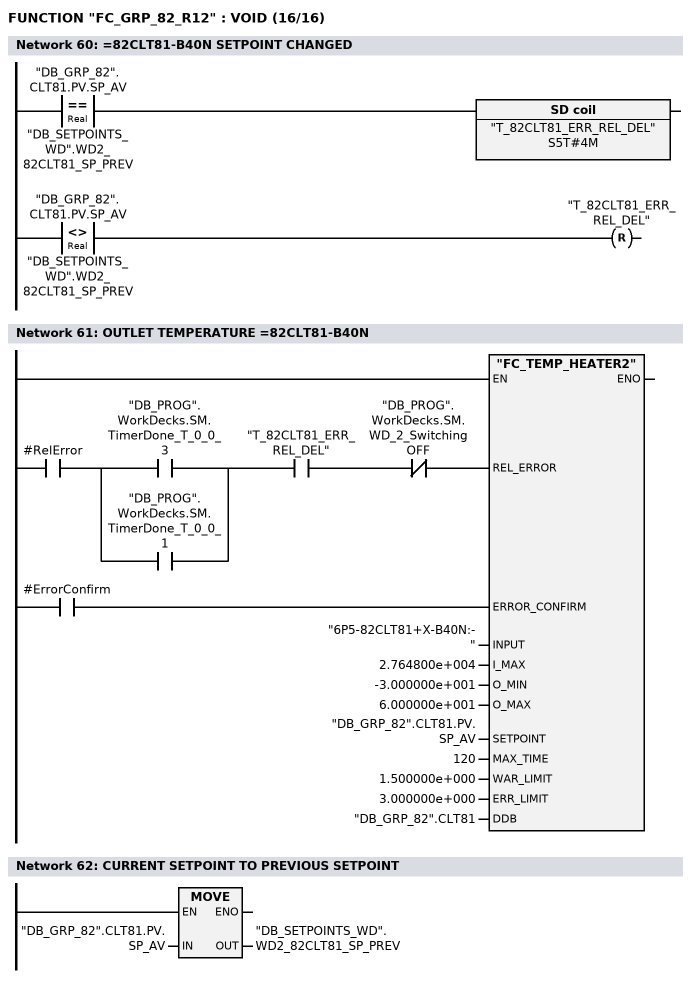
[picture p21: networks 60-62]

      U(    ;
      L     "DB_GRP_82".CLT81.PV.SP_AV;
      L     "DB_SETPOINTS_WD".WD2_82CLT81_SP_PREV;
      ==R   ;
      )     ;
      L     S5T#4M;
      SE    "T_82CLT81_ERR_REL_DEL";
      U(    ;
      L     "DB_GRP_82".CLT81.PV.SP_AV;
      L     "DB_SETPOINTS_WD".WD2_82CLT81_SP_PREV;
      <>R   ;
      )     ;
      R     "T_82CLT81_ERR_REL_DEL";
      NOP   0;
      NOP   0;
      NOP   0;
NETWORK
TITLE =OUTLET TEMPERATURE =82CLT81-B40N

      U     #RelError;
      U(    ;
      O     "DB_PROG".WorkDecks.SM.TimerDone_T_0_0_3;
      O     "DB_PROG".WorkDecks.SM.TimerDone_T_0_0_1;
      )     ;
      U     "T_82CLT81_ERR_REL_DEL";
      UN    "DB_PROG".WorkDecks.SM.WD_2_SwitchingOFF;
      =     L     16.0;
      BLD   103;
      U     #ErrorConfirm;
      =     L     16.1;
      BLD   103;
      CALL "FC_TEMP_HEATER2" (
           REL_ERROR                := L     16.0,
           ERROR_CONFIRM            := L     16.1,
           INPUT                    := "6P5-82CLT81+X-B40N:-",
           I_MAX                    := 2.764800e+004,
           O_MIN                    := -3.000000e+001,
           O_MAX                    := 6.000000e+001,
           SETPOINT                 := "DB_GRP_82".CLT81.PV.SP_AV,
           MAX_TIME                 := 120,
           WAR_LIMIT                := 1.500000e+000,
           ERR_LIMIT                := 3.000000e+000,
           DDB                      := "DB_GRP_82".CLT81);
      NOP   0;
NETWORK
TITLE =CURRENT SETPOINT TO PREVIOUS SETPOINT

      L     "DB_GRP_82".CLT81.PV.SP_AV;
      T     "DB_SETPOINTS_WD".WD2_82CLT81_SP_PREV;
      NOP   0;
NETWORK
TITLE =END

END_FUNCTION

